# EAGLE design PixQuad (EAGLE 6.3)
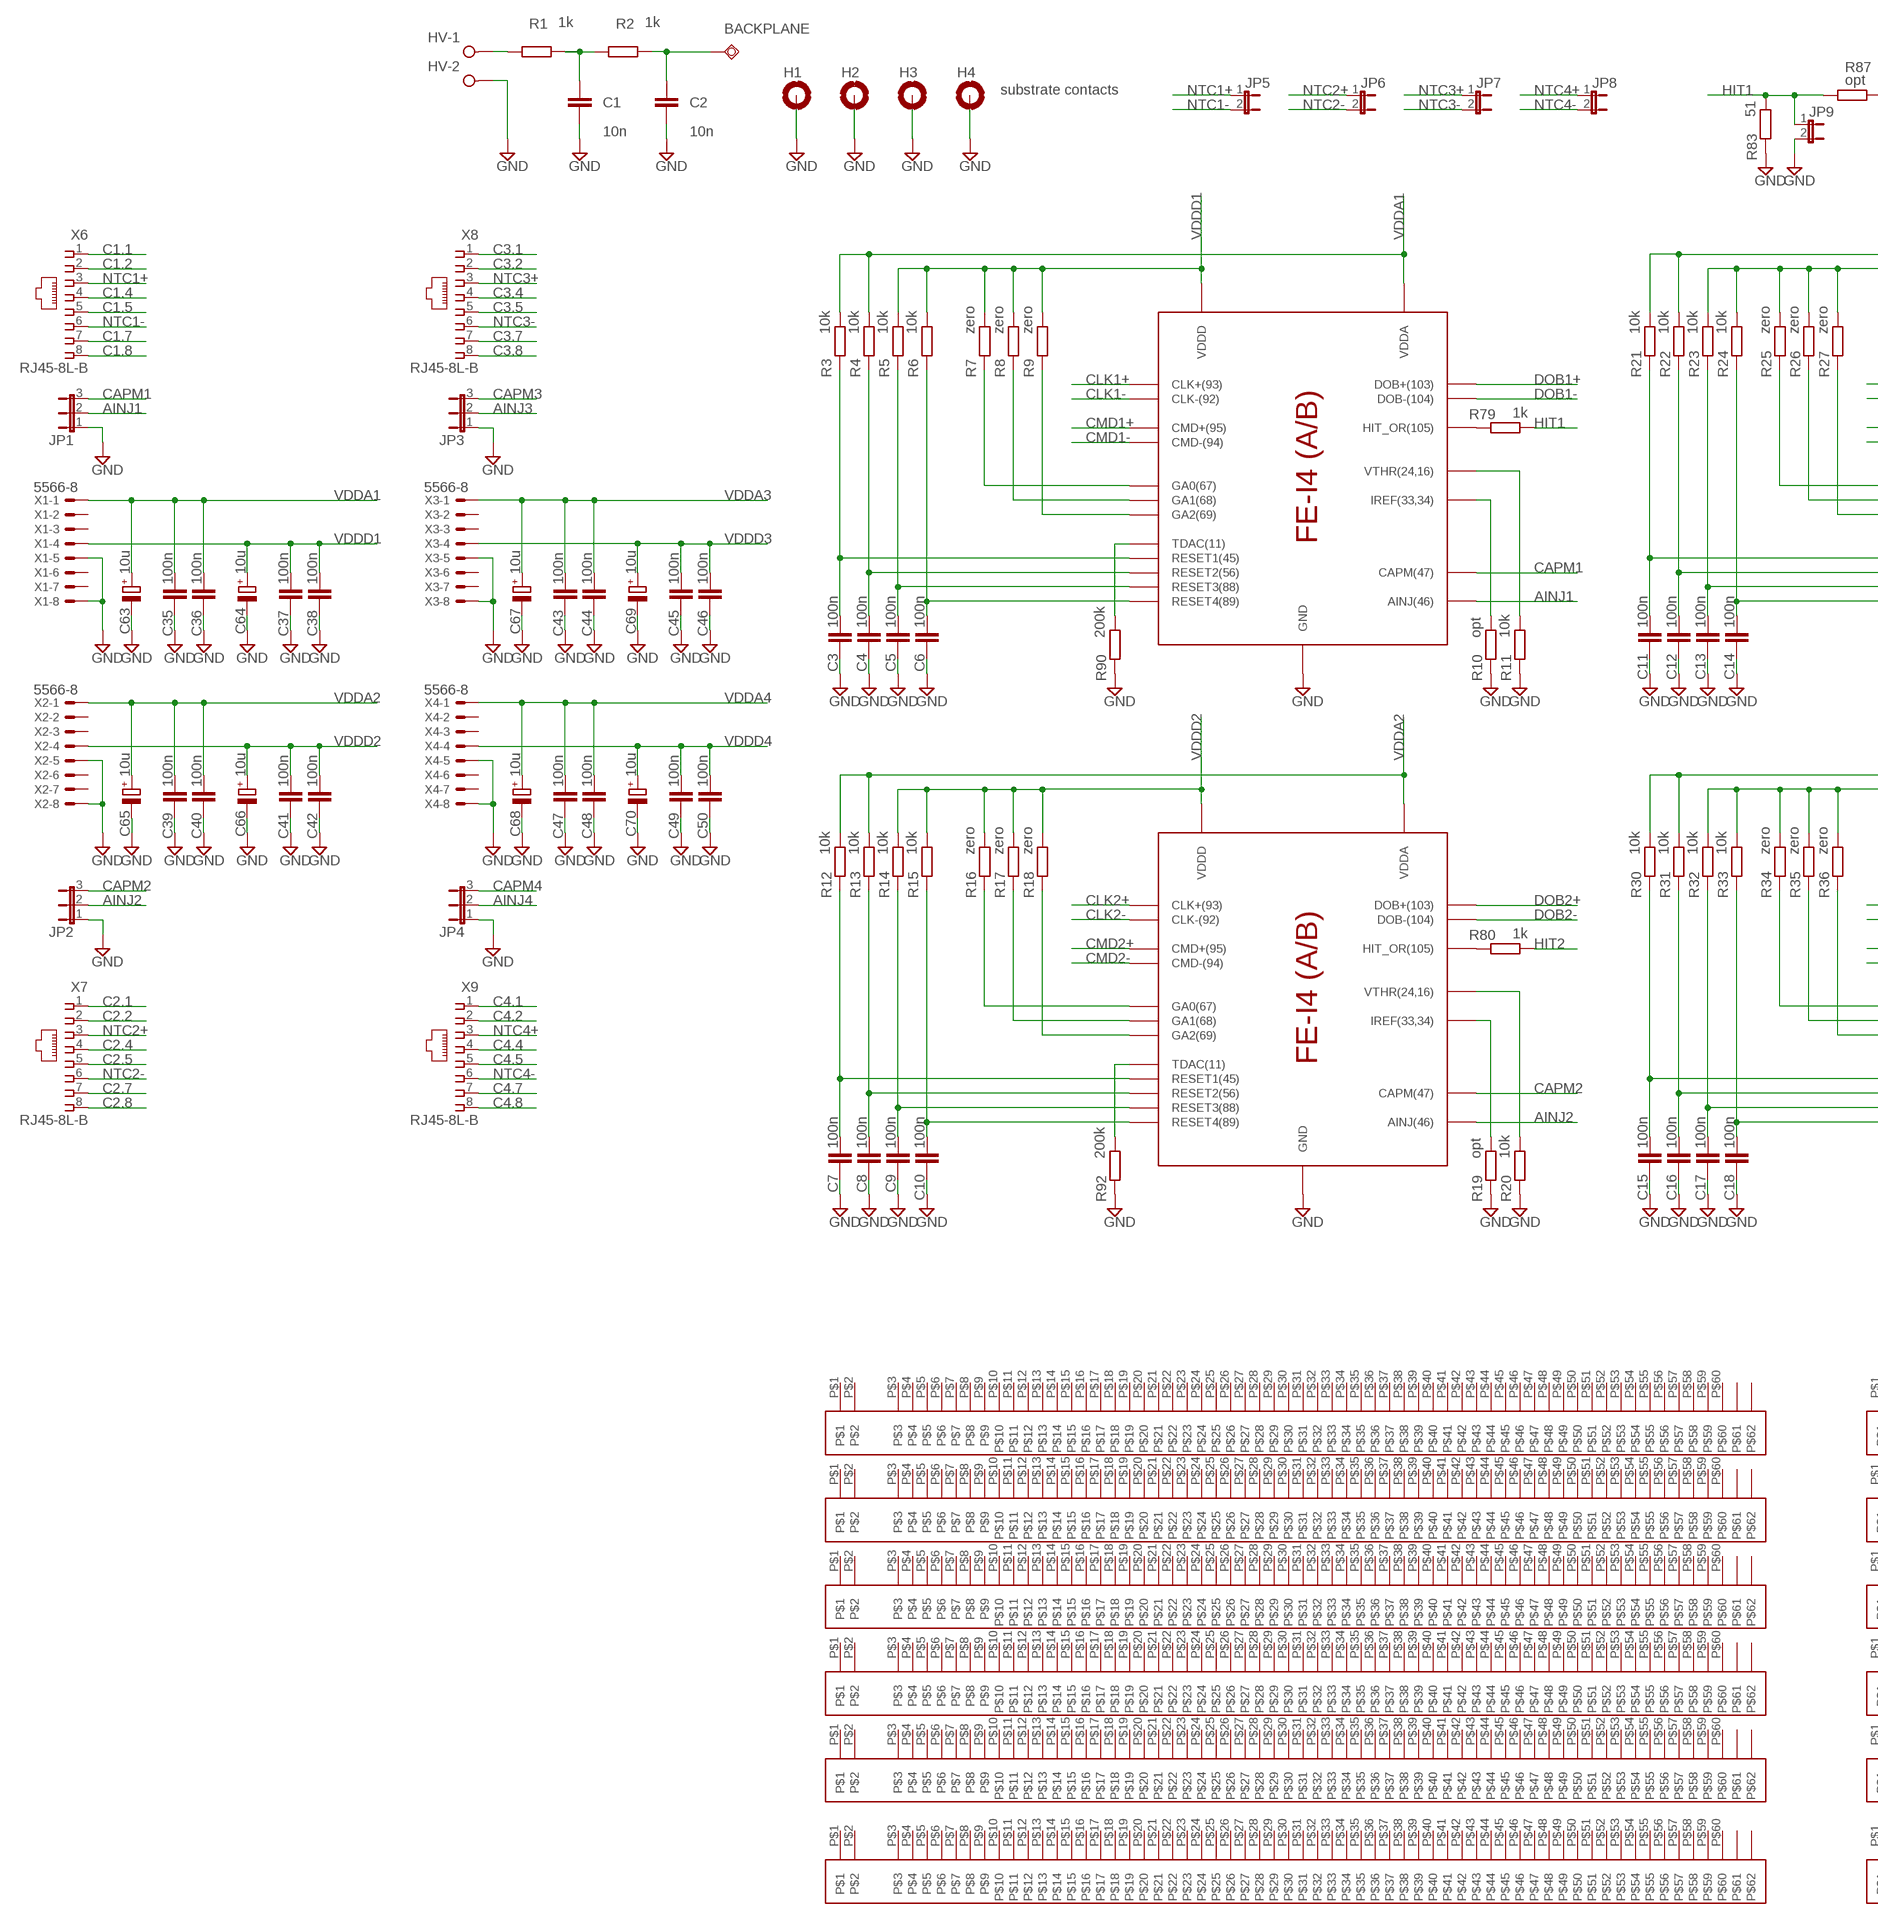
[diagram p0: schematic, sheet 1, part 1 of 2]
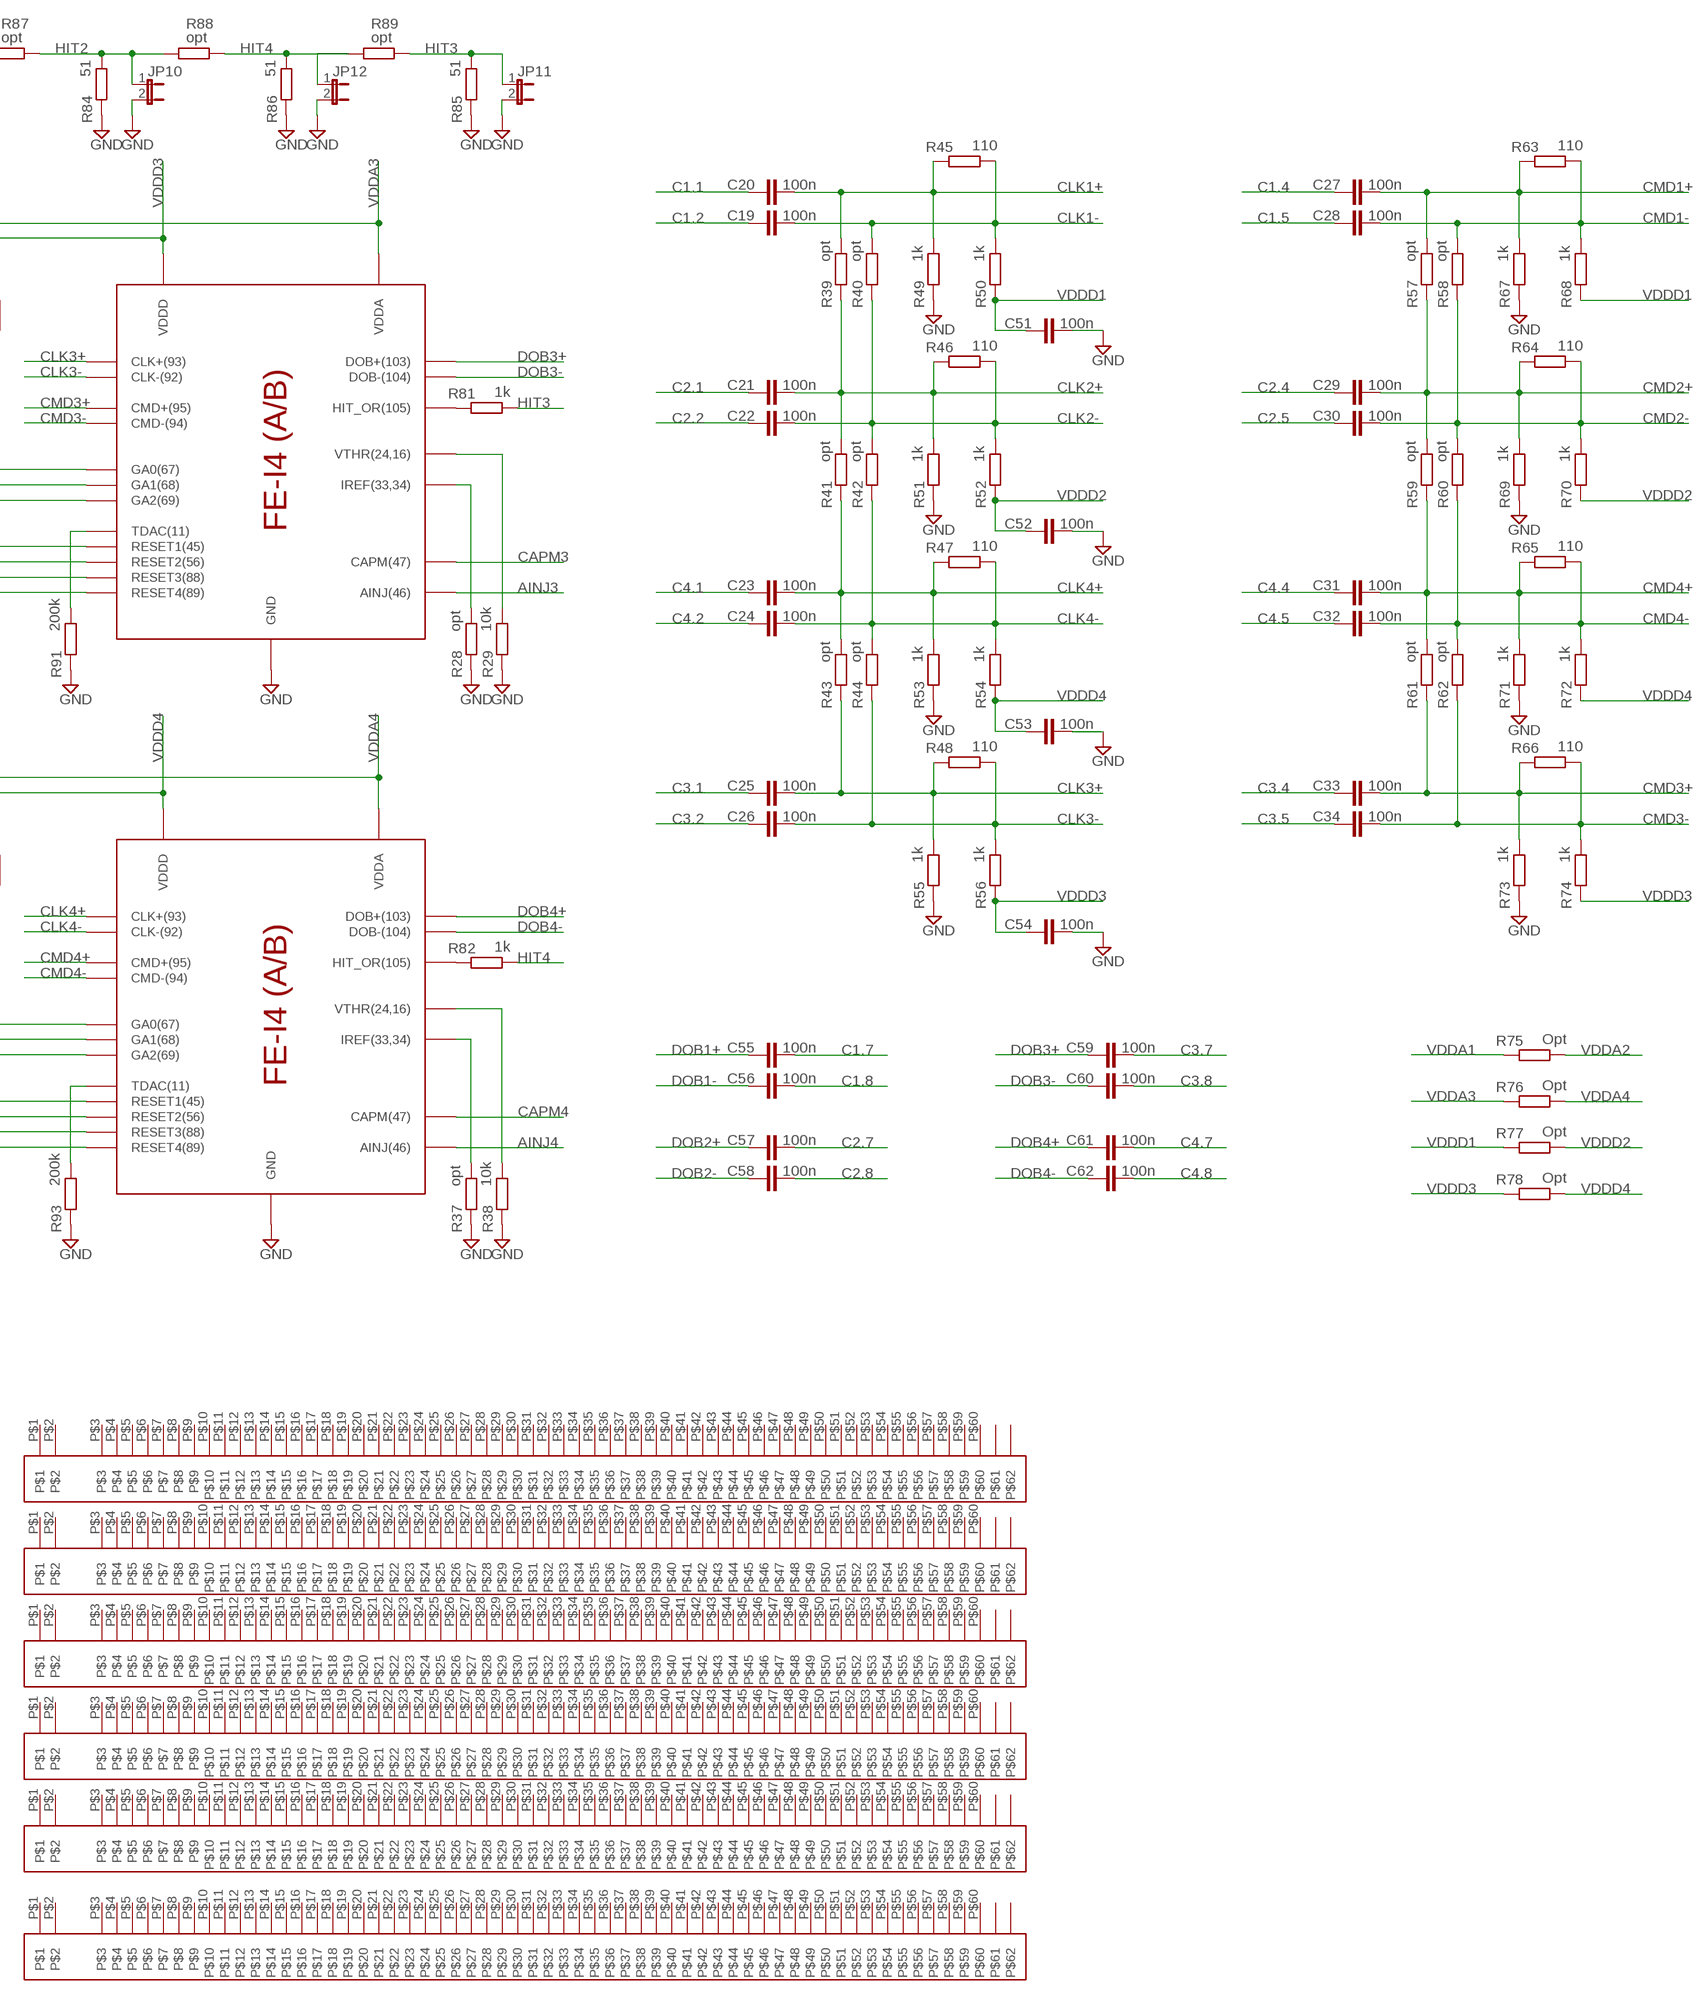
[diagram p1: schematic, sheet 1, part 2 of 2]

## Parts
BACKPLANE  TPSQTP20SQ  [TP20SQ]
C1  10n  C-EUC1210  [C1210]
C2  10n  C-EUC1210  [C1210]
C3  100n  C-EUC0402  [C0402]
C4  100n  C-EUC0402  [C0402]
C5  100n  C-EUC0402  [C0402]
C6  100n  C-EUC0402  [C0402]
C7  100n  C-EUC0402  [C0402]
C8  100n  C-EUC0402  [C0402]
C9  100n  C-EUC0402  [C0402]
C10  100n  C-EUC0402  [C0402]
C11  100n  C-EUC0402  [C0402]
C12  100n  C-EUC0402  [C0402]
C13  100n  C-EUC0402  [C0402]
C14  100n  C-EUC0402  [C0402]
C15  100n  C-EUC0402  [C0402]
C16  100n  C-EUC0402  [C0402]
C17  100n  C-EUC0402  [C0402]
C18  100n  C-EUC0402  [C0402]
C19  100n  C-EUC0402  [C0402]
C20  100n  C-EUC0402  [C0402]
C21  100n  C-EUC0402  [C0402]
C22  100n  C-EUC0402  [C0402]
C23  100n  C-EUC0402  [C0402]
C24  100n  C-EUC0402  [C0402]
C25  100n  C-EUC0402  [C0402]
C26  100n  C-EUC0402  [C0402]
C27  100n  C-EUC0402  [C0402]
C28  100n  C-EUC0402  [C0402]
C29  100n  C-EUC0402  [C0402]
C30  100n  C-EUC0402  [C0402]
C31  100n  C-EUC0402  [C0402]
C32  100n  C-EUC0402  [C0402]
C33  100n  C-EUC0402  [C0402]
C34  100n  C-EUC0402  [C0402]
C35  100n  C-EUC0402  [C0402]
C36  100n  C-EUC0402  [C0402]
C37  100n  C-EUC0402  [C0402]
C38  100n  C-EUC0402  [C0402]
C39  100n  C-EUC0402  [C0402]
C40  100n  C-EUC0402  [C0402]
C41  100n  C-EUC0402  [C0402]
C42  100n  C-EUC0402  [C0402]
C43  100n  C-EUC0402  [C0402]
C44  100n  C-EUC0402  [C0402]
C45  100n  C-EUC0402  [C0402]
C46  100n  C-EUC0402  [C0402]
C47  100n  C-EUC0402  [C0402]
C48  100n  C-EUC0402  [C0402]
C49  100n  C-EUC0402  [C0402]
C50  100n  C-EUC0402  [C0402]
C51  100n  C-EUC0402  [C0402]
C52  100n  C-EUC0402  [C0402]
C53  100n  C-EUC0402  [C0402]
C54  100n  C-EUC0402  [C0402]
C55  100n  C-EUC0402  [C0402]
C56  100n  C-EUC0402  [C0402]
C57  100n  C-EUC0402  [C0402]
C58  100n  C-EUC0402  [C0402]
C59  100n  C-EUC0402  [C0402]
C60  100n  C-EUC0402  [C0402]
C61  100n  C-EUC0402  [C0402]
C62  100n  C-EUC0402  [C0402]
C63  10u  CPOL-EUSMCA  [SMC_A]
C64  10u  CPOL-EUSMCA  [SMC_A]
C65  10u  CPOL-EUSMCA  [SMC_A]
C66  10u  CPOL-EUSMCA  [SMC_A]
C67  10u  CPOL-EUSMCA  [SMC_A]
C68  10u  CPOL-EUSMCA  [SMC_A]
C69  10u  CPOL-EUSMCA  [SMC_A]
C70  10u  CPOL-EUSMCA  [SMC_A]
H1  MOUNT-PAD-ROUND3.2  [3,2-PAD]
H2  MOUNT-PAD-ROUND3.2  [3,2-PAD]
H3  MOUNT-PAD-ROUND3.2  [3,2-PAD]
H4  substrate contacts  MOUNT-PAD-ROUND3.2  [3,2-PAD]
HV  W237-2N  [W237-2N]
JP1  JP2E  [JP2]
JP2  JP2E  [JP2]
JP3  JP2E  [JP2]
JP4  JP2E  [JP2]
JP5  JP1E  [JP1]
JP6  JP1E  [JP1]
JP7  JP1E  [JP1]
JP8  JP1E  [JP1]
JP9  JP1E  [JP1]
JP10  JP1E  [JP1]
JP11  JP1E  [JP1]
JP12  JP1E  [JP1]
R1  1k  R-EU_R1206  [R1206]
R2  1k  R-EU_R1206  [R1206]
R3  10k  R-EU_R0402  [R0402]
R4  10k  R-EU_R0402  [R0402]
R5  10k  R-EU_R0402  [R0402]
R6  10k  R-EU_R0402  [R0402]
R7  zero  R-EU_R0402  [R0402]
R8  zero  R-EU_R0402  [R0402]
R9  zero  R-EU_R0402  [R0402]
R10  opt  R-EU_R0402  [R0402]
R11  10k  R-EU_R0402  [R0402]
R12  10k  R-EU_R0402  [R0402]
R13  10k  R-EU_R0402  [R0402]
R14  10k  R-EU_R0402  [R0402]
R15  10k  R-EU_R0402  [R0402]
R16  zero  R-EU_R0402  [R0402]
R17  zero  R-EU_R0402  [R0402]
R18  zero  R-EU_R0402  [R0402]
R19  opt  R-EU_R0402  [R0402]
R20  10k  R-EU_R0402  [R0402]
R21  10k  R-EU_R0402  [R0402]
R22  10k  R-EU_R0402  [R0402]
R23  10k  R-EU_R0402  [R0402]
R24  10k  R-EU_R0402  [R0402]
R25  zero  R-EU_R0402  [R0402]
R26  zero  R-EU_R0402  [R0402]
R27  zero  R-EU_R0402  [R0402]
R28  opt  R-EU_R0402  [R0402]
R29  10k  R-EU_R0402  [R0402]
R30  10k  R-EU_R0402  [R0402]
R31  10k  R-EU_R0402  [R0402]
R32  10k  R-EU_R0402  [R0402]
R33  10k  R-EU_R0402  [R0402]
R34  zero  R-EU_R0402  [R0402]
R35  zero  R-EU_R0402  [R0402]
R36  zero  R-EU_R0402  [R0402]
R37  opt  R-EU_R0402  [R0402]
R38  10k  R-EU_R0402  [R0402]
R39  opt  R-EU_R0402  [R0402]
R40  opt  R-EU_R0402  [R0402]
R41  opt  R-EU_R0402  [R0402]
R42  opt  R-EU_R0402  [R0402]
R43  opt  R-EU_R0402  [R0402]
R44  opt  R-EU_R0402  [R0402]
R45  110  R-EU_R0402  [R0402]
R46  110  R-EU_R0402  [R0402]
R47  110  R-EU_R0402  [R0402]
R48  110  R-EU_R0402  [R0402]
R49  1k  R-EU_R0402  [R0402]
R50  1k  R-EU_R0402  [R0402]
R51  1k  R-EU_R0402  [R0402]
R52  1k  R-EU_R0402  [R0402]
R53  1k  R-EU_R0402  [R0402]
R54  1k  R-EU_R0402  [R0402]
R55  1k  R-EU_R0402  [R0402]
R56  1k  R-EU_R0402  [R0402]
R57  opt  R-EU_R0402  [R0402]
R58  opt  R-EU_R0402  [R0402]
R59  opt  R-EU_R0402  [R0402]
R60  opt  R-EU_R0402  [R0402]
R61  opt  R-EU_R0402  [R0402]
R62  opt  R-EU_R0402  [R0402]
R63  110  R-EU_R0402  [R0402]
R64  110  R-EU_R0402  [R0402]
R65  110  R-EU_R0402  [R0402]
R66  110  R-EU_R0402  [R0402]
R67  1k  R-EU_R0402  [R0402]
R68  1k  R-EU_R0402  [R0402]
R69  1k  R-EU_R0402  [R0402]
R70  1k  R-EU_R0402  [R0402]
R71  1k  R-EU_R0402  [R0402]
R72  1k  R-EU_R0402  [R0402]
R73  1k  R-EU_R0402  [R0402]
R74  1k  R-EU_R0402  [R0402]
R75  Opt  R-EU_R0402  [R0402]
R76  Opt  R-EU_R0402  [R0402]
R77  Opt  R-EU_R0402  [R0402]
R78  Opt  R-EU_R0402  [R0402]
R79  1k  R-EU_R0402  [R0402]
R80  1k  R-EU_R0402  [R0402]
R81  1k  R-EU_R0402  [R0402]
R82  1k  R-EU_R0402  [R0402]
R83  51  R-EU_R0402  [R0402]
R84  51  R-EU_R0402  [R0402]
R85  51  R-EU_R0402  [R0402]
R86  51  R-EU_R0402  [R0402]
R87  opt  R-EU_R0402  [R0402]
R88  opt  R-EU_R0402  [R0402]
R89  opt  R-EU_R0402  [R0402]
R90  200k  R-EU_R0402  [R0402]
R91  200k  R-EU_R0402  [R0402]
R92  200k  R-EU_R0402  [R0402]
R93  200k  R-EU_R0402  [R0402]
U$1  FE_I4ASIC  [FE-I4]
U$2  FE_I4ASIC  [FE-I4]
U$3  FE_I4ASIC  [FE-I4]
U$4  FE_I4ASIC  [FE-I4]
U$5  PA  [PA]
U$6  PA  [PA]
U$7  PA  [PA]
U$8  PA  [PA]
U$9  PA  [PA]
U$10  PA  [PA]
U$11  PA  [PA]
U$12  PA  [PA]
U$13  PA  [PA]
U$14  PA  [PA]
U$15  PA  [PA]
U$16  PA  [PA]
X1  5566-8  [5566-8]
X2  5566-8  [5566-8]
X3  5566-8  [5566-8]
X4  5566-8  [5566-8]
X6  RJ45-8L-B  [RJ45-NO-SHIELD]
X7  RJ45-8L-B  [RJ45-NO-SHIELD]
X8  RJ45-8L-B  [RJ45-NO-SHIELD]
X9  RJ45-8L-B  [RJ45-NO-SHIELD]

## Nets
AINJ1: JP1.2 U$1.AINJ(46)
AINJ2: JP2.2 U$2.AINJ(46)
AINJ3: JP3.2 U$3.AINJ(46)
AINJ4: JP4.2 U$4.AINJ(46)
C1.1: C20.2 X6.1
C1.2: C19.2 X6.2
C1.4: C27.2 X6.4
C1.5: C28.2 X6.5
C1.7: C55.1 X6.7
C1.8: C56.1 X6.8
C2.1: C21.2 X7.1
C2.2: C22.2 X7.2
C2.4: C29.2 X7.4
C2.5: C30.2 X7.5
C2.7: C57.1 X7.7
C2.8: C58.1 X7.8
C3.1: C25.2 X8.1
C3.2: C26.2 X8.2
C3.4: C33.2 X8.4
C3.5: C34.2 X8.5
C3.7: C59.1 X8.7
C3.8: C60.1 X8.8
C4.1: C23.2 X9.1
C4.2: C24.2 X9.2
C4.4: C31.2 X9.4
C4.5: C32.2 X9.5
C4.7: C61.1 X9.7
C4.8: C62.1 X9.8
CAPM1: JP1.3 U$1.CAPM(47)
CAPM2: JP2.3 U$2.CAPM(47)
CAPM3: JP3.3 U$3.CAPM(47)
CAPM4: JP4.3 U$4.CAPM(47)
CLK1+: C20.1 R39.2 R45.1 R49.2 U$1.CLK+(93)
CLK1-: C19.1 R40.2 R45.2 R50.2 U$1.CLK-(92)
CLK2+: C21.1 R39.1 R41.2 R46.1 R51.2 U$2.CLK+(93)
CLK2-: C22.1 R40.1 R42.2 R46.2 R52.2 U$2.CLK-(92)
CLK3+: C25.1 R43.1 R48.1 R55.2 U$3.CLK+(93)
CLK3-: C26.1 R44.1 R48.2 R56.2 U$3.CLK-(92)
CLK4+: C23.1 R41.1 R43.2 R47.1 R53.2 U$4.CLK+(93)
CLK4-: C24.1 R42.1 R44.2 R47.2 R54.2 U$4.CLK-(92)
CMD1+: C27.1 R57.2 R63.1 R67.2 U$1.CMD+(95)
CMD1-: C28.1 R58.2 R63.2 R68.2 U$1.CMD-(94)
CMD2+: C29.1 R57.1 R59.2 R64.1 R69.2 U$2.CMD+(95)
CMD2-: C30.1 R58.1 R60.2 R64.2 R70.2 U$2.CMD-(94)
CMD3+: C33.1 R61.1 R66.1 R73.2 U$3.CMD+(95)
CMD3-: C34.1 R62.1 R66.2 R74.2 U$3.CMD-(94)
CMD4+: C31.1 R59.1 R61.2 R65.1 R71.2 U$4.CMD+(95)
CMD4-: C32.1 R60.1 R62.2 R65.2 R72.2 U$4.CMD-(94)
DOB1+: C55.2 U$1.DOB+(103)
DOB1-: C56.2 U$1.DOB-(104)
DOB2+: C57.2 U$2.DOB+(103)
DOB2-: C58.2 U$2.DOB-(104)
DOB3+: C59.2 U$3.DOB+(103)
DOB3-: C60.2 U$3.DOB-(104)
DOB4+: C61.2 U$4.DOB+(103)
DOB4-: C62.2 U$4.DOB-(104)
GND: C1.2 C2.2 C3.2 C4.2 C5.2 C6.2 C7.2 C8.2 C9.2 C10.2 C11.2 C12.2 C13.2 C14.2 C15.2 C16.2 C17.2 C18.2 C35.2 C36.2 C37.2 C38.2 C39.2 C40.2 C41.2 C42.2 C43.2 C44.2 C45.2 C46.2 C47.2 C48.2 C49.2 C50.2 C51.1 C52.1 C53.1 C54.1 C63.- C64.- C65.- C66.- C67.- C68.- C69.- C70.- H1.B3,2(MOUNT) H2.B3,2(MOUNT) H3.B3,2(MOUNT) H4.B3,2(MOUNT) HV.2 JP1.1 JP2.1 JP3.1 JP4.1 JP9.2 JP10.2 JP11.2 JP12.2 R10.1 R11.1 R19.1 R20.1 R28.1 R29.1 R37.1 R38.1 R49.1 R51.1 R53.1 R55.1 R67.1 R69.1 R71.1 R73.1 R83.1 R84.1 R85.1 R86.1 R90.1 R91.1 R92.1 R93.1 U$1.GND U$2.GND U$3.GND U$4.GND X1.5 X1.8 X2.5 X2.8 X3.5 X3.8 X4.5 X4.8
HIT1: JP9.1 R79.2 R83.2 R87.2
HIT2: JP10.1 R80.2 R84.2 R87.1 R88.2
HIT3: JP11.1 R81.2 R85.2 R89.1
HIT4: JP12.1 R82.2 R86.2 R88.1 R89.2
N$1: BACKPLANE.TP C2.1 R2.2
N$2: C1.1 R1.2 R2.1
N$3: HV.1 R1.1
N$4: C3.1 R3.1 U$1.RESET1(45)
N$5: C4.1 R4.1 U$1.RESET2(56)
N$6: C5.1 R5.1 U$1.RESET3(88)
N$7: C6.1 R6.1 U$1.RESET4(89)
N$8: R7.1 U$1.GA0(67)
N$9: R8.1 U$1.GA1(68)
N$10: R9.1 U$1.GA2(69)
N$11: R10.2 U$1.IREF(33,34)
N$12: R11.2 U$1.VTHR(24,16)
N$13: R79.1 U$1.P$1(HIT_OR(105))
N$14: R16.1 U$2.GA0(67)
N$15: R17.1 U$2.GA1(68)
N$16: R18.1 U$2.GA2(69)
N$17: C7.1 R12.1 U$2.RESET1(45)
N$18: C8.1 R13.1 U$2.RESET2(56)
N$19: C9.1 R14.1 U$2.RESET3(88)
N$20: C10.1 R15.1 U$2.RESET4(89)
N$21: R80.1 U$2.P$1(HIT_OR(105))
N$22: R81.1 U$3.P$1(HIT_OR(105))
N$23: R82.1 U$4.P$1(HIT_OR(105))
N$24: R90.2 U$1.TDAC(11)
N$25: R19.2 U$2.IREF(33,34)
N$26: R20.2 U$2.VTHR(24,16)
N$27: R91.2 U$3.TDAC(11)
N$28: R92.2 U$2.TDAC(11)
N$29: R93.2 U$4.TDAC(11)
N$50: R27.1 U$3.GA2(69)
N$56: R28.2 U$3.IREF(33,34)
N$57: R26.1 U$3.GA1(68)
N$58: R25.1 U$3.GA0(67)
N$59: C11.1 R21.1 U$3.RESET1(45)
N$60: C12.1 R22.1 U$3.RESET2(56)
N$61: C13.1 R23.1 U$3.RESET3(88)
N$62: C14.1 R24.1 U$3.RESET4(89)
N$64: R29.2 U$3.VTHR(24,16)
N$73: R34.1 U$4.GA0(67)
N$74: R35.1 U$4.GA1(68)
N$75: R36.1 U$4.GA2(69)
N$76: C15.1 R30.1 U$4.RESET1(45)
N$77: C16.1 R31.1 U$4.RESET2(56)
N$78: C17.1 R32.1 U$4.RESET3(88)
N$79: C18.1 R33.1 U$4.RESET4(89)
N$80: R37.2 U$4.IREF(33,34)
N$81: R38.2 U$4.VTHR(24,16)
NTC1+: JP5.1 X6.3
NTC1-: JP5.2 X6.6
NTC2+: JP6.1 X7.3
NTC2-: JP6.2 X7.6
NTC3+: JP7.1 X8.3
NTC3-: JP7.2 X8.6
NTC4+: JP8.1 X9.3
NTC4-: JP8.2 X9.6
VDDA1: C35.1 C36.1 C63.+ R3.2 R4.2 R75.1 U$1.VDDA X1.1
VDDA2: C39.1 C40.1 C65.+ R12.2 R13.2 R75.2 U$2.VDDA X2.1
VDDA3: C43.1 C44.1 C67.+ R21.2 R22.2 R76.1 U$3.VDDA X3.1
VDDA4: C47.1 C48.1 C68.+ R30.2 R31.2 R76.2 U$4.VDDA X4.1
VDDD1: C37.1 C38.1 C51.2 C64.+ R5.2 R6.2 R7.2 R8.2 R9.2 R50.1 R68.1 R77.1 U$1.VDDD X1.4
VDDD2: C41.1 C42.1 C52.2 C66.+ R14.2 R15.2 R16.2 R17.2 R18.2 R52.1 R70.1 R77.2 U$2.VDDD X2.4
VDDD3: C45.1 C46.1 C54.2 C69.+ R23.2 R24.2 R25.2 R26.2 R27.2 R56.1 R74.1 R78.1 U$3.VDDD X3.4
VDDD4: C49.1 C50.1 C53.2 C70.+ R32.2 R33.2 R34.2 R35.2 R36.2 R54.1 R72.1 R78.2 U$4.VDDD X4.4
Unconnected: U$5.P$1 U$5.P$2 U$5.P$3 U$5.P$4 U$5.P$5 U$5.P$6 U$5.P$7 U$5.P$8 U$5.P$9 U$5.P$10 U$5.P$11 U$5.P$12 U$5.P$13 U$5.P$14 U$5.P$15 U$5.P$16 U$5.P$17 U$5.P$18 U$5.P$19 U$5.P$20 U$5.P$21 U$5.P$22 U$5.P$23 U$5.P$24 U$5.P$25 U$5.P$26 U$5.P$27 U$5.P$28 U$5.P$29 U$5.P$30 U$5.P$31 U$5.P$32 U$5.P$33 U$5.P$34 U$5.P$35 U$5.P$36 U$5.P$37 U$5.P$38 U$5.P$39 U$5.P$40 U$5.P$41 U$5.P$42 U$5.P$43 U$5.P$44 U$5.P$45 U$5.P$46 U$5.P$47 U$5.P$48 U$5.P$49 U$5.P$50 U$5.P$51 U$5.P$52 U$5.P$53 U$5.P$54 U$5.P$55 U$5.P$56 U$5.P$57 U$5.P$58 U$5.P$59 U$5.P$60 U$5.P$61 U$5.P$62 U$6.P$1 U$6.P$2 U$6.P$3 U$6.P$4 U$6.P$5 U$6.P$6 U$6.P$7 U$6.P$8 U$6.P$9 U$6.P$10 U$6.P$11 U$6.P$12 U$6.P$13 U$6.P$14 U$6.P$15 U$6.P$16 U$6.P$17 U$6.P$18 U$6.P$19 U$6.P$20 U$6.P$21 U$6.P$22 U$6.P$23 U$6.P$24 U$6.P$25 U$6.P$26 U$6.P$27 U$6.P$28 U$6.P$29 U$6.P$30 U$6.P$31 U$6.P$32 U$6.P$33 U$6.P$34 U$6.P$35 U$6.P$36 U$6.P$37 U$6.P$38 U$6.P$39 U$6.P$40 U$6.P$41 U$6.P$42 U$6.P$43 U$6.P$44 U$6.P$45 U$6.P$46 U$6.P$47 U$6.P$48 U$6.P$49 U$6.P$50 U$6.P$51 U$6.P$52 U$6.P$53 U$6.P$54 U$6.P$55 U$6.P$56 U$6.P$57 U$6.P$58 U$6.P$59 U$6.P$60 U$6.P$61 U$6.P$62 U$7.P$1 U$7.P$2 U$7.P$3 U$7.P$4 U$7.P$5 U$7.P$6 U$7.P$7 U$7.P$8 U$7.P$9 U$7.P$10 U$7.P$11 U$7.P$12 U$7.P$13 U$7.P$14 U$7.P$15 U$7.P$16 U$7.P$17 U$7.P$18 U$7.P$19 U$7.P$20 U$7.P$21 U$7.P$22 U$7.P$23 U$7.P$24 U$7.P$25 U$7.P$26 U$7.P$27 U$7.P$28 U$7.P$29 U$7.P$30 U$7.P$31 U$7.P$32 U$7.P$33 U$7.P$34 U$7.P$35 U$7.P$36 U$7.P$37 U$7.P$38 U$7.P$39 U$7.P$40 U$7.P$41 U$7.P$42 U$7.P$43 U$7.P$44 U$7.P$45 U$7.P$46 U$7.P$47 U$7.P$48 U$7.P$49 U$7.P$50 U$7.P$51 U$7.P$52 U$7.P$53 U$7.P$54 U$7.P$55 U$7.P$56 U$7.P$57 U$7.P$58 U$7.P$59 U$7.P$60 U$7.P$61 U$7.P$62 U$8.P$1 U$8.P$2 U$8.P$3 U$8.P$4 U$8.P$5 U$8.P$6 U$8.P$7 U$8.P$8 U$8.P$9 U$8.P$10 U$8.P$11 U$8.P$12 U$8.P$13 U$8.P$14 U$8.P$15 U$8.P$16 U$8.P$17 U$8.P$18 U$8.P$19 U$8.P$20 U$8.P$21 U$8.P$22 U$8.P$23 U$8.P$24 U$8.P$25 U$8.P$26 U$8.P$27 U$8.P$28 U$8.P$29 U$8.P$30 U$8.P$31 U$8.P$32 U$8.P$33 U$8.P$34 U$8.P$35 U$8.P$36 U$8.P$37 U$8.P$38 U$8.P$39 U$8.P$40 U$8.P$41 U$8.P$42 U$8.P$43 U$8.P$44 U$8.P$45 U$8.P$46 U$8.P$47 U$8.P$48 U$8.P$49 U$8.P$50 U$8.P$51 U$8.P$52 U$8.P$53 U$8.P$54 U$8.P$55 U$8.P$56 U$8.P$57 U$8.P$58 U$8.P$59 U$8.P$60 U$8.P$61 U$8.P$62 U$9.P$1 U$9.P$2 U$9.P$3 U$9.P$4 U$9.P$5 U$9.P$6 U$9.P$7 U$9.P$8 U$9.P$9 U$9.P$10 U$9.P$11 U$9.P$12 U$9.P$13 U$9.P$14 U$9.P$15 U$9.P$16 U$9.P$17 U$9.P$18 U$9.P$19 U$9.P$20 U$9.P$21 U$9.P$22 U$9.P$23 U$9.P$24 U$9.P$25 U$9.P$26 U$9.P$27 U$9.P$28 U$9.P$29 U$9.P$30 U$9.P$31 U$9.P$32 U$9.P$33 U$9.P$34 U$9.P$35 U$9.P$36 U$9.P$37 U$9.P$38 U$9.P$39 U$9.P$40 U$9.P$41 U$9.P$42 U$9.P$43 U$9.P$44 U$9.P$45 U$9.P$46 U$9.P$47 U$9.P$48 U$9.P$49 U$9.P$50 U$9.P$51 U$9.P$52 U$9.P$53 U$9.P$54 U$9.P$55 U$9.P$56 U$9.P$57 U$9.P$58 U$9.P$59 U$9.P$60 U$9.P$61 U$9.P$62 U$10.P$1 U$10.P$2 U$10.P$3 U$10.P$4 U$10.P$5 U$10.P$6 U$10.P$7 U$10.P$8 U$10.P$9 U$10.P$10 U$10.P$11 U$10.P$12 U$10.P$13 U$10.P$14 U$10.P$15 U$10.P$16 U$10.P$17 U$10.P$18 U$10.P$19 U$10.P$20 U$10.P$21 U$10.P$22 U$10.P$23 U$10.P$24 U$10.P$25 U$10.P$26 U$10.P$27 U$10.P$28 U$10.P$29 U$10.P$30 U$10.P$31 U$10.P$32 U$10.P$33 U$10.P$34 U$10.P$35 U$10.P$36 U$10.P$37 U$10.P$38 U$10.P$39 U$10.P$40 U$10.P$41 U$10.P$42 U$10.P$43 U$10.P$44 U$10.P$45 U$10.P$46 U$10.P$47 U$10.P$48 U$10.P$49 U$10.P$50 U$10.P$51 U$10.P$52 U$10.P$53 U$10.P$54 U$10.P$55 U$10.P$56 U$10.P$57 U$10.P$58 U$10.P$59 U$10.P$60 U$10.P$61 U$10.P$62 U$11.P$1 U$11.P$2 U$11.P$3 U$11.P$4 U$11.P$5 U$11.P$6 U$11.P$7 U$11.P$8 U$11.P$9 U$11.P$10 U$11.P$11 U$11.P$12 U$11.P$13 U$11.P$14 U$11.P$15 U$11.P$16 U$11.P$17 U$11.P$18 U$11.P$19 U$11.P$20 U$11.P$21 U$11.P$22 U$11.P$23 U$11.P$24 U$11.P$25 U$11.P$26 U$11.P$27 U$11.P$28 U$11.P$29 U$11.P$30 U$11.P$31 U$11.P$32 U$11.P$33 U$11.P$34 U$11.P$35 U$11.P$36 U$11.P$37 U$11.P$38 U$11.P$39 U$11.P$40 U$11.P$41 U$11.P$42 U$11.P$43 U$11.P$44 U$11.P$45 U$11.P$46 U$11.P$47 U$11.P$48 U$11.P$49 U$11.P$50 U$11.P$51 U$11.P$52 U$11.P$53 U$11.P$54 U$11.P$55 U$11.P$56 U$11.P$57 U$11.P$58 U$11.P$59 U$11.P$60 U$11.P$61 U$11.P$62 U$12.P$1 U$12.P$2 U$12.P$3 U$12.P$4 U$12.P$5 U$12.P$6 U$12.P$7 U$12.P$8 U$12.P$9 U$12.P$10 U$12.P$11 U$12.P$12 U$12.P$13 U$12.P$14 U$12.P$15 U$12.P$16 U$12.P$17 U$12.P$18 U$12.P$19 U$12.P$20 U$12.P$21 U$12.P$22 U$12.P$23 U$12.P$24 U$12.P$25 U$12.P$26 U$12.P$27 U$12.P$28 U$12.P$29 U$12.P$30 U$12.P$31 U$12.P$32 U$12.P$33 U$12.P$34 U$12.P$35 U$12.P$36 U$12.P$37 U$12.P$38 U$12.P$39 U$12.P$40 U$12.P$41 U$12.P$42 U$12.P$43 U$12.P$44 U$12.P$45 U$12.P$46 U$12.P$47 U$12.P$48 U$12.P$49 U$12.P$50 U$12.P$51 U$12.P$52 U$12.P$53 U$12.P$54 U$12.P$55 U$12.P$56 U$12.P$57 U$12.P$58 U$12.P$59 U$12.P$60 U$12.P$61 U$12.P$62 U$13.P$1 U$13.P$2 U$13.P$3 U$13.P$4 U$13.P$5 U$13.P$6 U$13.P$7 U$13.P$8 U$13.P$9 U$13.P$10 U$13.P$11 U$13.P$12 U$13.P$13 U$13.P$14 U$13.P$15 U$13.P$16 U$13.P$17 U$13.P$18 U$13.P$19 U$13.P$20 U$13.P$21 U$13.P$22 U$13.P$23 U$13.P$24 U$13.P$25 U$13.P$26 U$13.P$27 U$13.P$28 U$13.P$29 U$13.P$30 U$13.P$31 U$13.P$32 U$13.P$33 U$13.P$34 U$13.P$35 U$13.P$36 U$13.P$37 U$13.P$38 U$13.P$39 U$13.P$40 U$13.P$41 U$13.P$42 U$13.P$43 U$13.P$44 U$13.P$45 U$13.P$46 U$13.P$47 U$13.P$48 U$13.P$49 U$13.P$50 U$13.P$51 U$13.P$52 U$13.P$53 U$13.P$54 U$13.P$55 U$13.P$56 U$13.P$57 U$13.P$58 U$13.P$59 U$13.P$60 U$13.P$61 U$13.P$62 U$14.P$1 U$14.P$2 U$14.P$3 U$14.P$4 U$14.P$5 U$14.P$6 U$14.P$7 U$14.P$8 U$14.P$9 U$14.P$10 U$14.P$11 U$14.P$12 U$14.P$13 U$14.P$14 U$14.P$15 U$14.P$16 U$14.P$17 U$14.P$18 U$14.P$19 U$14.P$20 U$14.P$21 U$14.P$22 U$14.P$23 U$14.P$24 U$14.P$25 U$14.P$26 U$14.P$27 U$14.P$28 U$14.P$29 U$14.P$30 U$14.P$31 U$14.P$32 U$14.P$33 U$14.P$34 U$14.P$35 U$14.P$36 U$14.P$37 U$14.P$38 U$14.P$39 U$14.P$40 U$14.P$41 U$14.P$42 U$14.P$43 U$14.P$44 U$14.P$45 U$14.P$46 U$14.P$47 U$14.P$48 U$14.P$49 U$14.P$50 U$14.P$51 U$14.P$52 U$14.P$53 U$14.P$54 U$14.P$55 U$14.P$56 U$14.P$57 U$14.P$58 U$14.P$59 U$14.P$60 U$14.P$61 U$14.P$62 U$15.P$1 U$15.P$2 U$15.P$3 U$15.P$4 U$15.P$5 U$15.P$6 U$15.P$7 U$15.P$8 U$15.P$9 U$15.P$10 U$15.P$11 U$15.P$12 U$15.P$13 U$15.P$14 U$15.P$15 U$15.P$16 U$15.P$17 U$15.P$18 U$15.P$19 U$15.P$20 U$15.P$21 U$15.P$22 U$15.P$23 U$15.P$24 U$15.P$25 U$15.P$26 U$15.P$27 U$15.P$28 U$15.P$29 U$15.P$30 U$15.P$31 U$15.P$32 U$15.P$33 U$15.P$34 U$15.P$35 U$15.P$36 U$15.P$37 U$15.P$38 U$15.P$39 U$15.P$40 U$15.P$41 U$15.P$42 U$15.P$43 U$15.P$44 U$15.P$45 U$15.P$46 U$15.P$47 U$15.P$48 U$15.P$49 U$15.P$50 U$15.P$51 U$15.P$52 U$15.P$53 U$15.P$54 U$15.P$55 U$15.P$56 U$15.P$57 U$15.P$58 U$15.P$59 U$15.P$60 U$15.P$61 U$15.P$62 U$16.P$1 U$16.P$2 U$16.P$3 U$16.P$4 U$16.P$5 U$16.P$6 U$16.P$7 U$16.P$8 U$16.P$9 U$16.P$10 U$16.P$11 U$16.P$12 U$16.P$13 U$16.P$14 U$16.P$15 U$16.P$16 U$16.P$17 U$16.P$18 U$16.P$19 U$16.P$20 U$16.P$21 U$16.P$22 U$16.P$23 U$16.P$24 U$16.P$25 U$16.P$26 U$16.P$27 U$16.P$28 U$16.P$29 U$16.P$30 U$16.P$31 U$16.P$32 U$16.P$33 U$16.P$34 U$16.P$35 U$16.P$36 U$16.P$37 U$16.P$38 U$16.P$39 U$16.P$40 U$16.P$41 U$16.P$42 U$16.P$43 U$16.P$44 U$16.P$45 U$16.P$46 U$16.P$47 U$16.P$48 U$16.P$49 U$16.P$50 U$16.P$51 U$16.P$52 U$16.P$53 U$16.P$54 U$16.P$55 U$16.P$56 U$16.P$57 U$16.P$58 U$16.P$59 U$16.P$60 U$16.P$61 U$16.P$62 X1.2 X1.3 X1.6 X1.7 X2.2 X2.3 X2.6 X2.7 X3.2 X3.3 X3.6 X3.7 X4.2 X4.3 X4.6 X4.7

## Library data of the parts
BACKPLANE = testpad:TPSQ: Test pad
C1-C62 = rcl:C-EU: CAPACITOR, European symbol
C63-C70 = rcl:CPOL-EU: POLARIZED CAPACITOR, European symbol
H1-H4 = holes:MOUNT-PAD-ROUND: MOUNTING PAD, round
HV = con-wago-508:W237-2N: WAGO SREW CLAMP; OC_FARNELL: unknown; OC_NEWARK: unknown
JP1-JP4 = jumper:JP2E: JUMPER
JP5-JP12 = jumper:JP1E: JUMPER
R1-R93 = rcl:R-EU_: RESISTOR, European symbol
U$1-U$4 = FE-I4:FE_I4
U$5-U$16 = FE-I4:PA
X1-X4 = FE-I4:5566-8: Mini FIT connector 8 pol Source: http://www.molex.com; OC_FARNELL: unknown; OC_NEWARK: unknown
X6-X9 = con-tycoelectronics:RJ45: CORCOM Modular RJ Jacks No Shield Source: www.tycoelectronics.com .. ENG_DS_1654001_1099_RJ_L_0507.pdf; MF: TYCO ELECTRONICS; MPN: RJ45-8L-B; OC_FARNELL: 1279843; OC_NEWARK: 52K4445

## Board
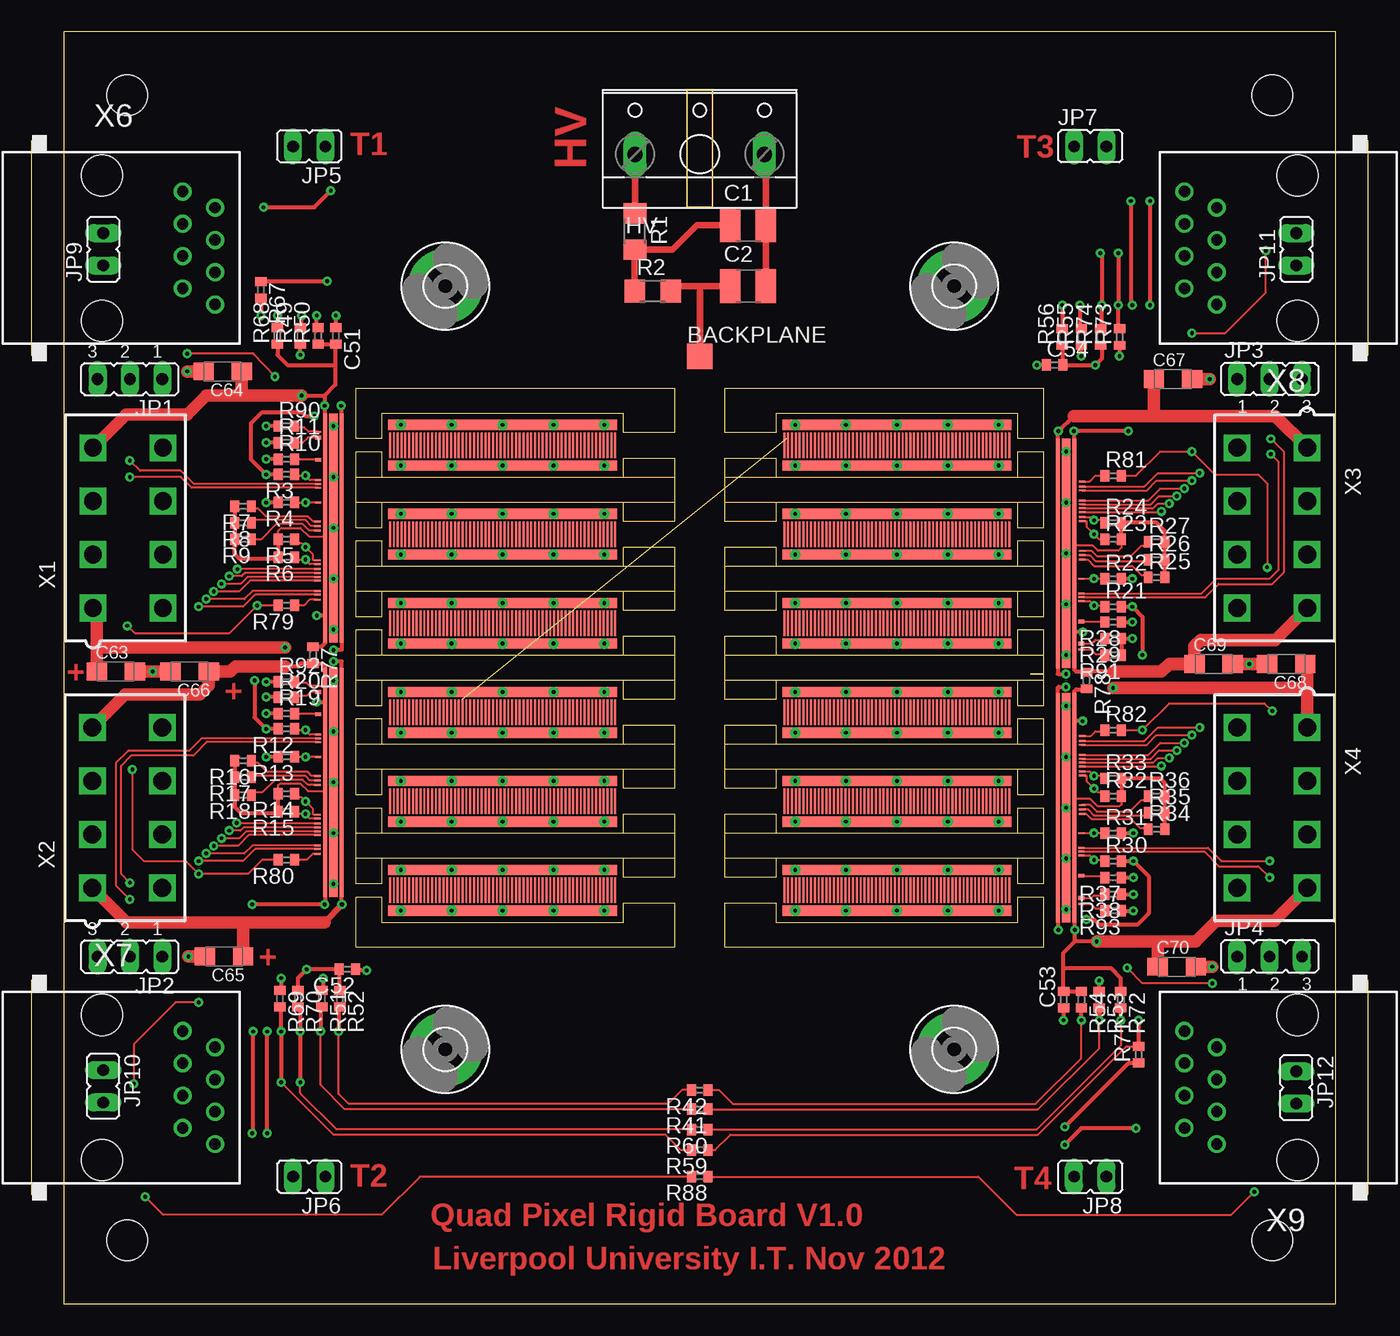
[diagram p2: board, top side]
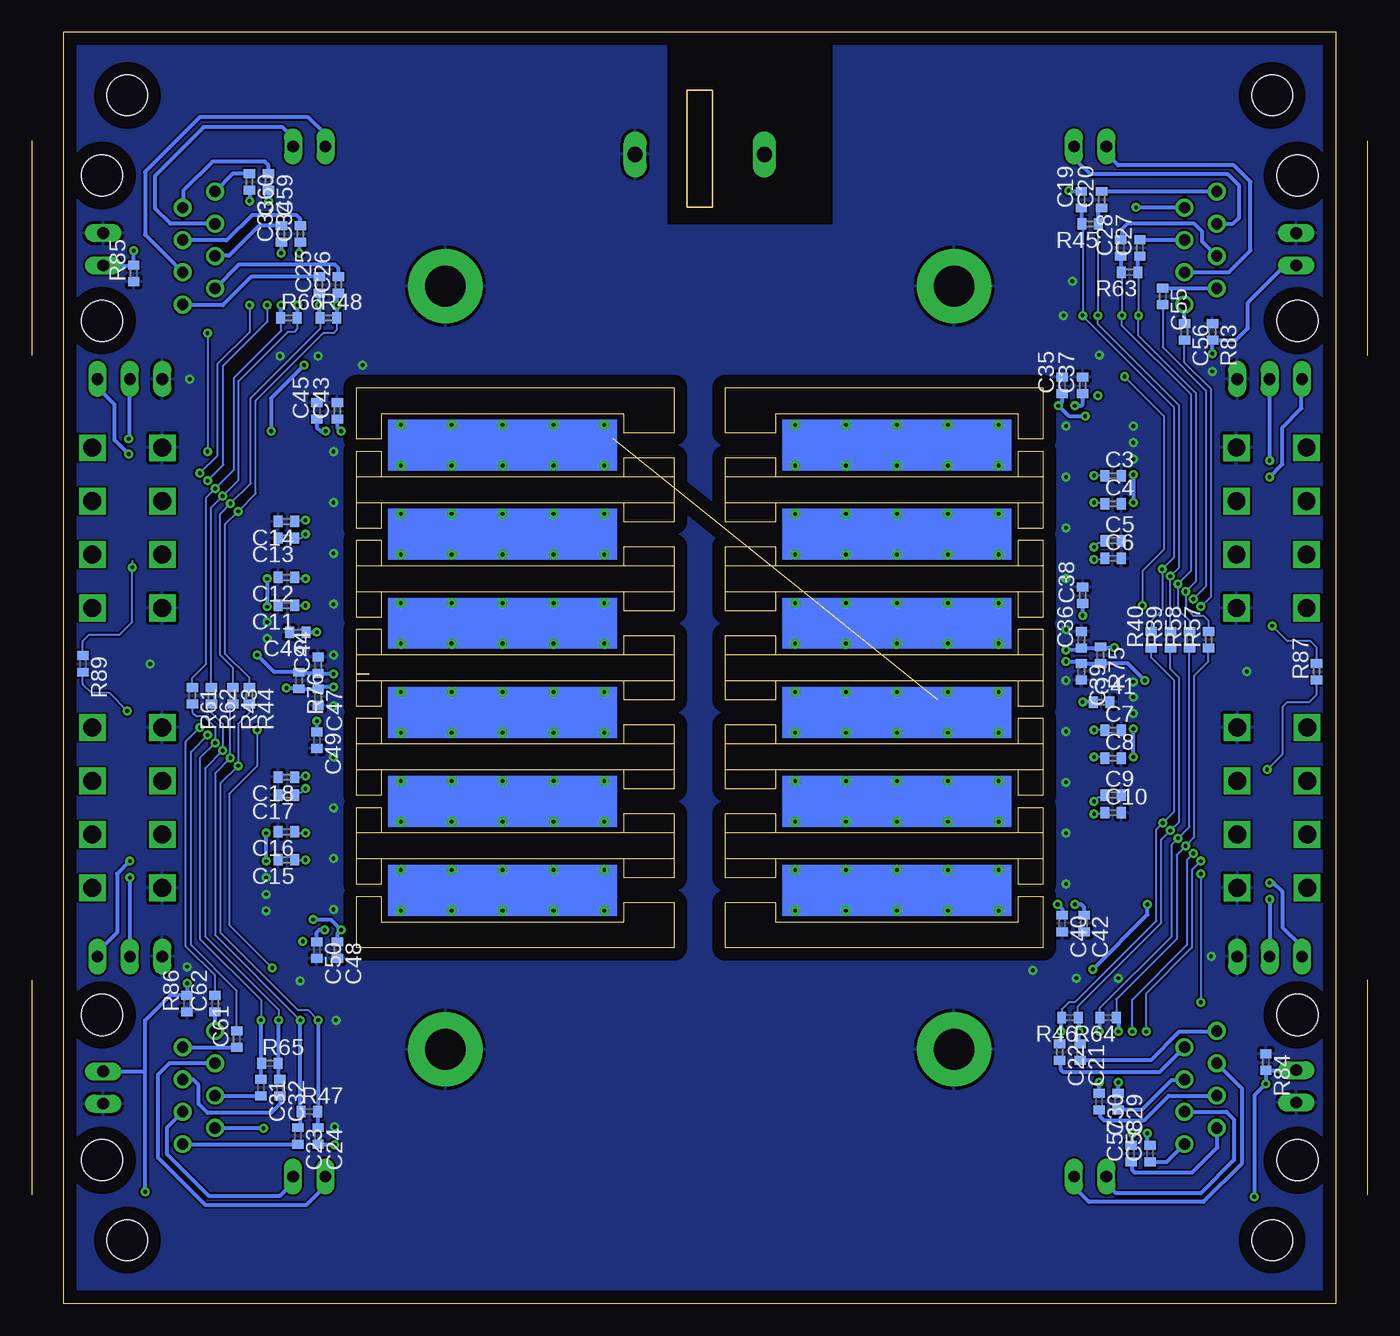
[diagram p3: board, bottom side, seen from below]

Size 105.02 x 100 mm. Coordinates in mm from the lower left corner, seen from the top.
Outline: 2.51,0 102.51,0 102.51,100 2.51,100 2.51,0
Copper layers (1+2*15+16): Top 0.035mm / dielectric 1.5mm / Route2 0.035mm / dielectric 0.15mm / Route15 0.035mm / dielectric 0.2mm / Bottom 0.035mm
Design rules "default *": minimum track width 10mil, minimum drill 24mil, track to track 6mil, track to pad 6mil, pad to pad 6mil, via to via 6mil, smd to smd 6mil, copper to edge 40mil, drill to drill 8mil, minimum pad ring 10mil, minimum via ring 8mil, stop-mask expansion 4mil, vias tented up to drill 0mil, thermal gap 10mil
Holes 3.2 mm at 7.51,5 7.51,95 97.51,95 97.51,5

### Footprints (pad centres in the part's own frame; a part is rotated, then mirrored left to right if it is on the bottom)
TP20SQ = smd 2 x 2: TP 0,0
C1210 = smd 1.6 x 2.7: 1 -1.4,0; 2 1.4,0
C0402 = smd 0.7 x 0.9: 1 -0.65,0; 2 0.65,0
SMC_A = smd 1.6 x 1.4: + -1.5,0; - 1.5,0
3,2-PAD = drill 3.2 pad 5.842: B3,2 0,0
W237-2N = drill 1.194 long: 1 -5.08,-0.635; 2 5.08,-0.635
JP2 = drill 0.914 long: 1 -2.54,0; 2 0,0; 3 2.54,0
JP1 = drill 0.914 long: 1 0,-1.27; 2 0,1.27
R1206 = smd 1.6 x 1.803: 1 -1.422,0; 2 1.422,0
R0402 = smd 0.7 x 0.9: 1 -0.65,0; 2 0.65,0
FE-I4 = smd 0.15 x 0.5: AINJ(46) -4.45,-2; CAPM(47) -4.15,-2; CLK+(93) 2.55,-2.05; CLK-(92) 2.25,-2.05; CMD+(95) 3.15,-2.05; CMD-(94) 2.85,-2.05; DOB+(103) 3.95,-2.05; DOB-(104) 4.25,-2.05; GA0(67) -1.5,-2.05; GA1(68) -1.15,-2.05; GA2(69) -0.8,-2.05; P$1 4.65,-2.05; RESET1(45) -4.75,-2; RESET2(56) -3,-2; RESET3(88) 1.55,-2.05; RESET4(89) 1.85,-2.05; TDAC(11) -8.55,-2 | smd 18 x 0.7: GND -1,-0.8 | smd 0.3 x 0.5: IREF(33,34) -6.35,-2; VTHR(24,16) -8.1,-2 | smd 18 x 0.3: VDDA -1,-0.15; VDDD -1,-1.45
PA = smd 18 x 0.8: P$1 -9,-0.4; P$2 -9,-3.6 | smd 0.15 x 2: P$3 -17.85,-2; P$4 -17.55,-2; P$5 -17.25,-2; P$6 -16.95,-2; P$7 -16.65,-2; P$8 -16.35,-2; P$9 -16.05,-2; P$10 -15.75,-2; P$11 -15.45,-2; P$12 -15.15,-2; P$13 -14.85,-2; P$14 -14.55,-2; P$15 -14.25,-2; P$16 -13.95,-2; P$17 -13.65,-2; P$18 -13.35,-2; P$19 -13.05,-2; P$20 -12.75,-2; P$21 -12.45,-2; P$22 -12.15,-2; P$23 -11.85,-2; P$24 -11.55,-2; P$25 -11.25,-2; P$26 -10.95,-2; P$27 -10.65,-2; P$28 -10.35,-2; P$29 -10.05,-2; P$30 -9.75,-2; P$31 -9.45,-2; P$32 -9.15,-2; P$33 -8.85,-2; P$34 -8.55,-2; P$35 -8.25,-2; P$36 -7.95,-2; P$37 -7.65,-2; P$38 -7.35,-2; P$39 -7.05,-2; P$40 -6.75,-2; P$41 -6.45,-2; P$42 -6.15,-2; P$43 -5.85,-2; P$44 -5.55,-2; P$45 -5.25,-2; P$46 -4.95,-2; P$47 -4.65,-2; P$48 -4.35,-2; P$49 -4.05,-2; P$50 -3.75,-2; P$51 -3.45,-2; P$52 -3.15,-2; P$53 -2.85,-2; P$54 -2.55,-2; P$55 -2.25,-2; P$56 -1.95,-2; P$57 -1.65,-2; P$58 -1.35,-2; P$59 -1.05,-2; P$60 -0.75,-2; P$71 -0.45,-2; P$72 -0.15,-2 | drill 0.3 pad 0.7: P$61 -17,-0.4; P$62 -13,-0.4; P$63 -9,-0.4; P$64 -5,-0.4; P$65 -1,-0.4; P$66 -17,-3.6; P$67 -13,-3.6; P$68 -9,-3.6; P$69 -5,-3.6; P$70 -1,-3.6
5566-8 = drill 1.4 square: 1 6.3,-2.75; 2 2.1,-2.75; 3 -2.1,-2.75; 4 -6.3,-2.75; 5 6.3,2.75; 6 2.1,2.75; 7 -2.1,2.75; 8 -6.3,2.75
RJ45-NO-SHIELD = drill 0.9 pad 1.4: 1 -4.445,6.35; 2 -3.175,8.89; 3 -1.905,6.35; 4 -0.635,8.89; 5 0.635,6.35; 6 1.905,8.89; 7 3.175,6.35; 8 4.445,8.89 | hole 3.251: -5.715,0; 5.715,0

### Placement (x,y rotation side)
BACKPLANE  52.51,74.5 0 top
C1  56.31,84.8 0 top
C2  56.31,80 0 top
C3  20.01,65.1 0 bottom
C4  20.01,62.9 0 bottom
C5  20.01,60 0 bottom
C6  20.01,58.6 0 bottom
C7  20.01,45.1 0 bottom
C8  20.01,42.9 0 bottom
C9  20.01,40 0 bottom
C10  20.01,38.6 0 bottom
C11  85.01,54.9 180 bottom
C12  85.01,57.1 180 bottom
C13  85.01,60.2 180 bottom
C14  85.01,61.5 180 bottom
C15  85.01,34.9 180 bottom
C16  85.01,37.1 180 bottom
C17  85.01,40 180 bottom
C18  85.01,41.4 180 bottom
C19  22.51,86.8 90 bottom
C20  20.91,86.8 90 bottom
C21  22.61,19.8 270 bottom
C22  24.21,19.8 270 bottom
C23  84.11,13.2 270 bottom
C24  82.51,13.2 270 bottom
C25  82.41,80.1 90 bottom
C26  80.91,80.1 90 bottom
C27  17.91,83 90 bottom
C28  19.41,83 90 bottom
C29  19.61,15.9 270 bottom
C30  21.11,15.9 270 bottom
C31  87.01,17 270 bottom
C32  85.51,17 270 bottom
C33  85.41,84.1 90 bottom
C34  83.91,84.1 90 bottom
C35  24.01,72.2 90 bottom
C36  22.51,52.2 90 bottom
C37  22.41,72.2 90 bottom
C38  22.41,55.7 90 bottom
C39  22.51,49.7 270 bottom
C40  24.01,29.9 270 bottom
C41  20.91,47.3 0 bottom
C42  22.31,29.9 270 bottom
C43  81.01,70.2 90 bottom
C44  82.51,50.2 90 bottom
C45  82.61,70.2 90 bottom
C46  84.11,52.8 180 bottom
C47  82.51,47.7 270 bottom
C48  81.01,27.8 270 bottom
C49  82.61,44.3 270 bottom
C50  82.61,27.8 270 bottom
C51  23.91,76.1 270 top
C52  24.81,26.3 180 top
C53  81.11,23.9 90 top
C54  80.41,73.8 0 top
C55  16.11,79.2 270 bottom
C56  14.41,76.4 270 bottom
C57  18.61,11.8 90 bottom
C58  17.11,11.8 90 bottom
C59  86.41,88.2 270 bottom
C60  87.91,88.2 270 bottom
C61  88.91,20.8 90 bottom
C62  90.61,23.6 90 bottom
C63  6.61,49.7 0 top
C64  15.01,73.3 180 top
C65  15.11,27.3 180 top
C66  12.41,49.7 180 top
C67  89.71,72.7 0 top
C68  98.61,50.3 180 top
C69  92.91,50.3 0 top
C70  90.01,26.5 0 top
H1  32.51,80 0 top
H2  32.51,20 0 top
H3  72.51,80 0 top
H4  72.51,20 0 top
HV  52.51,91 0 top
JP1  7.71,72.7 180 top
JP2  7.71,27.3 180 top
JP3  97.31,72.7 0 top
JP4  97.31,27.3 0 top
JP5  21.81,91 90 top
JP6  21.81,10 90 top
JP7  83.21,91 270 top
JP8  83.21,10 90 top
JP9  5.61,82.9 0 top
JP10  5.61,17.1 180 top
JP11  99.41,82.9 0 top
JP12  99.41,17 180 top
R1  47.41,84.3 270 top
R2  48.81,79.6 0 top
R3  20.01,65.2 180 top
R4  20.01,63 180 top
R5  20.01,60.1 180 top
R6  20.01,58.7 180 top
R7  16.61,62.7 180 top
R8  16.61,61.4 180 top
R9  16.61,60.1 180 top
R10  20.01,66.4 0 top
R11  20.01,67.7 0 top
R12  20.01,45.2 180 top
R13  20.01,43 180 top
R14  20.01,40.1 180 top
R15  20.01,38.7 180 top
R16  16.61,42.7 180 top
R17  16.61,41.4 180 top
R18  16.61,40 180 top
R19  20.01,46.4 0 top
R20  20.01,47.7 0 top
R21  85.01,54.8 0 top
R22  85.01,57 0 top
R23  85.01,60.1 0 top
R24  85.01,61.4 0 top
R25  88.41,57.1 0 top
R26  88.41,58.5 0 top
R27  88.41,59.9 0 top
R28  85.01,53.6 180 top
R29  85.01,52.3 180 top
R30  85.01,34.8 0 top
R31  85.01,37 0 top
R32  85.01,39.9 0 top
R33  85.01,41.3 0 top
R34  88.41,37.3 0 top
R35  88.41,38.6 0 top
R36  88.41,39.9 0 top
R37  85.01,33.5 180 top
R38  85.01,32.2 180 top
R39  15.51,52.2 90 bottom
R40  17.01,52.2 90 bottom
R41  52.51,15.3 180 top
R42  52.51,16.8 180 top
R43  89.21,47.8 270 bottom
R44  87.91,47.8 270 bottom
R45  21.81,84.9 180 bottom
R46  23.41,22.5 180 bottom
R47  83.21,15.1 0 bottom
R48  81.71,77.5 0 bottom
R49  21.11,76.1 90 top
R50  22.51,76.1 90 top
R51  22.81,24 270 top
R52  24.21,24 270 top
R53  83.91,23.9 270 top
R54  82.51,23.9 270 top
R55  82.51,76 90 top
R56  81.01,76 90 top
R57  12.51,52.2 90 bottom
R58  14.01,52.2 90 bottom
R59  52.51,12.1 180 top
R60  52.51,13.7 180 top
R61  92.41,47.8 270 bottom
R62  90.91,47.8 270 bottom
R63  18.71,81.1 180 bottom
R64  20.41,22.5 180 bottom
R65  86.31,18.9 0 bottom
R66  84.81,77.5 0 bottom
R67  18.01,79.7 270 top
R68  19.31,76.1 90 top
R69  19.51,24 270 top
R70  20.91,24 270 top
R71  87.01,19.6 90 top
R72  85.61,23.9 270 top
R73  85.51,76 90 top
R74  84.01,76 90 top
R75  21.01,51 270 bottom
R76  84.01,49 270 bottom
R77  22.11,51 270 top
R78  82.91,49 270 top
R79  20.01,54.9 180 top
R80  20.01,34.9 180 top
R81  85.01,65.1 0 top
R82  85.01,45.1 0 top
R83  12.21,76.4 270 bottom
R84  8.01,19 270 bottom
R85  97.01,81 90 bottom
R86  92.81,23.6 90 bottom
R87  4.01,49.7 90 bottom
R88  52.51,10 180 top
R89  101.01,50.3 270 bottom
R90  20.01,69 0 top
R91  85.01,51 180 top
R92  20.01,48.9 0 top
R93  85.01,30.9 180 top
U$1  24.51,60 270 top
U$2  24.51,40 270 top
U$3  80.51,60 90 top
U$4  80.51,40 90 top
U$5  28.01,65.5 180 top
U$6  28.01,58.5 180 top
U$7  28.01,44.5 180 top
U$8  28.01,51.5 180 top
U$9  28.01,37.5 180 top
U$10  28.01,30.5 180 top
U$11  59.01,65.5 180 top
U$12  59.01,58.5 180 top
U$13  59.01,51.5 180 top
U$14  59.01,44.5 180 top
U$15  59.01,37.5 180 top
U$16  59.01,30.5 180 top
X1  7.56,61 270 top
X2  7.51,39 270 top
X3  97.51,61 90 top
X4  97.51,39 90 top
X6  5.51,83 270 top
X7  5.51,17 270 top
X8  99.51,83 90 top
X9  99.51,17 90 top

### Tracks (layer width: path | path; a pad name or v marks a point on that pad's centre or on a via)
AINJ1  (via drill 0.3)
  Top 0.15: U$1.AINJ(46) 12.76,64.45 11.71,65.5 8.51,65.5 v7.71,66.3
  Bottom 0.3: v7.71,66.3 JP1.2
AINJ2  (via drill 0.3)
  Top 0.15: U$2.AINJ(46) 13.36,44.45 12.41,43.5 7.61,43.5 6.61,42.5 6.61,32.9 v7.71,31.8
  Bottom 0.3: v7.71,31.8 JP2.2
AINJ3  (via drill 0.3)
  Top 0.15: U$3.AINJ(46) 92.26,55.55 93.31,56.6 97.51,56.6 98.41,57.5 98.41,67 v97.41,68
  Bottom 0.3: v97.41,68 97.31,68.1 JP3.2
AINJ4  (via drill 0.3)
  Top 0.15: U$4.AINJ(46) 92.16,35.55 93.31,34.4 96.41,34.4 v97.31,33.5
  Bottom 0.3: v97.31,33.5 JP4.2
C1.1
  Bottom 0.3: X6.1 C20.2
C1.2  (via drill 0.3)
  Top 0.3: v18.21,86.2 22.21,86.2 v23.51,87.5
  Bottom 0.3: X6.2 18.19,86.17 v18.21,86.2 | C19.2 23.46,87.45 v23.51,87.5
C1.4
  Bottom 0.3: X6.4 17.9,83.64 C27.2
C1.5
  Bottom 0.3: X6.5 13.01,83.52 13.01,84.3 13.61,84.9 18.91,84.9 19.31,84.5 19.31,83.75 C28.2
C1.7
  Bottom 0.15: 16.09,79.83 C55.1
  Bottom 0.3: X6.7 16.09,79.83
C1.8
  Bottom 0.15: 14.41,78.55 X6.8
  Bottom 0.3: C56.1 14.41,78.55
C2.1
  Bottom 0.3: C21.2 17.06,19.15 14.81,21.4 11.91,21.4 X7.1
C2.2
  Bottom 0.3: X7.2 16.38,18.2 23.91,18.2 24.11,18.4 24.11,19.05 C22.2
C2.4
  Bottom 0.3: C29.2 19.56,15.3 17.71,15.3 15.41,17.6 14.44,17.6 X7.4
C2.5
  Bottom 0.3: X7.5 15.65,16.37 17.61,14.4 20.71,14.4 21.01,14.7 21.01,15.15 C30.2
C2.7
  Bottom 0.3: X7.7 11.81,13.78 11.81,12.3 13.81,10.3 18.31,10.3 18.51,10.5 18.51,11.05 C57.1
C2.8
  Bottom 0.3: C58.1 15.81,11.15 X7.8
C3.1
  Bottom 0.3: C25.2 87.76,80.75 90.01,78.5 93.11,78.5 X8.1
C3.2
  Bottom 0.3: C26.2 80.91,81.4 81.21,81.7 88.75,81.7 X8.2
C3.4
  Bottom 0.3: C33.2 87.16,84.75 89.51,82.4 90.59,82.4 X8.4
C3.5
  Bottom 0.3: C34.2 83.91,85.3 84.21,85.6 87.71,85.6 89.71,83.6 93.13,83.6 X8.5
C3.7
  Bottom 0.3: C59.1 86.41,89.5 86.71,89.8 90.81,89.8 93.11,87.5 93.11,86.22 X8.7
C3.8
  Bottom 0.3: C60.1 89.22,88.85 X8.8
C4.1
  Bottom 0.3: X9.1 C23.2
C4.2  (via drill 0.3)
  Top 0.3: v86.81,13.8 82.51,13.8 v81.21,12.5
  Bottom 0.3: X9.2 86.84,13.82 v86.81,13.8 | v81.21,12.5 82.46,12.5 C24.2
C4.4
  Bottom 0.3: X9.4 87.03,16.37 C31.2
C4.5
  Bottom 0.3: C32.2 85.51,15.7 86.21,15 91.21,15 91.91,15.7 91.91,17.2 92.35,17.63 X9.5
C4.7
  Bottom 0.3: X9.7 88.94,20.18 C61.1
C4.8
  Bottom 0.3: X9.8 C62.1
CAPM1  (via drill 0.3)
  Top 0.15: U$1.CAPM(47) 12.56,64.15 11.71,65 v7.71,65
  Bottom 0.3: v7.71,65 6.71,66 6.71,68.9 5.21,70.4 5.21,72.66 JP1.3
CAPM2  (via drill 0.3)
  Top 0.15: U$2.CAPM(47) 13.76,44.15 12.71,43.1 7.81,43.1 7.01,42.3 7.01,33.8 v7.71,33.1
  Bottom 0.3: v7.71,33.1 7.41,33.1 6.71,32.4 6.71,29.6 5.31,28.2 5.31,27.44 JP2.3
CAPM3  (via drill 0.3)
  Top 0.15: U$3.CAPM(47) 91.96,55.85 93.11,57 97.31,57 98.01,57.7 98.01,66.2 v97.41,66.8
  Bottom 0.3: v97.41,66.8 98.51,67.9 98.51,70.7 99.85,72.04 JP3.3
CAPM4  (via drill 0.3)
  Top 0.15: U$4.CAPM(47) 92.46,35.85 93.51,34.8 v97.31,34.8
  Bottom 0.3: v97.31,34.8 98.31,33.8 98.31,29.2 99.85,27.66 JP4.3
CLK1+  (via drill 0.3)
  Top 0.15: U$1.CLK+(93) 16.76,57.45 16.51,57.2 v15.51,57.2
  Top 0.3: R49.2 21.21,76.75 v21.21,77.7
  Bottom 0.15: R39.2 v15.51,57.2 14.81,57.9 14.81,70.6 21.21,77 v21.21,77.7 21.21,84.85 R45.1
  Bottom 0.3: R45.1 21.16,85.9 C20.1
CLK1-  (via drill 0.3)
  Top 0.15: U$1.CLK-(92) v16.16,57.75
  Top 0.3: R50.2 22.41,76.75 v22.41,77.7
  Bottom 0.15: R40.2 17.01,53.7 16.16,54.55 v16.16,57.75 15.21,58.7 15.21,70.45 22.41,77.65 v22.41,77.7 22.41,84.85 R45.2
  Bottom 0.3: R45.2 22.46,86.1 C19.1
CLK2+  (via drill 0.3)
  Top 0.15: U$2.CLK+(93) 16.66,37.45 16.41,37.2 v15.51,37.2 | v22.71,21.4 22.71,17.2 24.61,15.3 R41.2
  Top 0.3: R51.2 22.71,23.25 v22.71,21.4
  Bottom 0.15: R39.1 15.51,49.9 14.81,49.2 14.81,37.9 v15.51,37.2 16.21,36.5 16.21,29.95 R51.2 22.81,22.55 R46.1
  Bottom 0.3: 22.81,22.5 R46.1 22.71,22.5 v22.71,21.4 22.71,20.55 C21.1
CLK2-  (via drill 0.3)
  Top 0.15: U$2.CLK-(92) 16.16,37.75 v16.11,37.8 | R42.2 51.11,16.8 50.01,15.7 24.91,15.7 24.11,16.5 v24.11,21.4
  Top 0.3: R52.2 24.11,23.25 v24.11,21.4
  Bottom 0.15: v16.11,37.8 15.21,38.7 15.21,49 17.01,50.8 R40.1 | v16.11,37.8 16.21,37.7 | 24.11,22.55 R46.2 24.06,23.15 23.51,23.7 23.01,23.7 16.61,30.1 16.61,37.3 v16.11,37.8
  Bottom 0.3: R46.2 24.11,22.5 v24.11,21.4 24.11,20.55 C22.1
CLK3+  (via drill 0.3)
  Top 0.15: U$3.CLK+(93) 88.16,62.55 88.51,62.9 v89.41,62.9
  Top 0.3: v82.41,78.5 82.41,76.75 R55.2
  Bottom 0.15: R43.1 89.21,50 90.21,51 90.21,62.1 v89.41,62.9 87.81,64.5 87.81,71.2 82.36,76.65 R48.1
  Bottom 0.3: C25.1 v82.41,78.5 82.41,77.55 R48.1
CLK3-  (via drill 0.3)
  Top 0.15: U$3.CLK-(92) 88.76,62.25 v88.81,62.3
  Top 0.3: v81.01,78.5 R56.2
  Bottom 0.15: R44.1 87.91,49.2 89.81,51.1 89.81,61.3 v88.81,62.3 87.41,63.7 87.41,71 82.11,76.3 81.31,76.3 81.06,76.55 R48.2
  Bottom 0.3: C26.1 81.01,79.35 v81.01,78.5 81.01,77.55 R48.2
CLK4+  (via drill 0.3)
  Top 0.15: U$4.CLK+(93) 88.16,42.55 88.51,42.9 v89.41,42.9 | v83.91,22.3 83.91,20.1 79.11,15.3 R41.1
  Top 0.3: R53.2 v83.91,22.3
  Bottom 0.15: v83.91,22.3 90.61,29 90.61,41.7 v89.41,42.9 89.41,46.95 R43.2
  Bottom 0.3: v83.91,22.3 83.91,15.25 R47.1 83.91,15.05 83.91,14.05 C23.1 83.86,13.85
CLK4-  (via drill 0.3)
  Top 0.15: U$4.CLK-(92) 88.76,42.25 v88.81,42.3 | R42.1 54.01,16.8 55.11,15.7 78.91,15.7 82.51,19.3 v82.51,22.3
  Top 0.3: v82.51,22.3 R54.2
  Bottom 0.15: v82.51,22.3 83.31,23.1 84.11,23.1 90.21,29.2 90.21,40.9 v88.81,42.3 88.81,45.6 87.91,46.5 R44.2
  Bottom 0.3: C24.1 82.56,13.85 R47.2 82.51,15.1 v82.51,22.3
CMD1+  (via drill 0.3)
  Top 0.15: U$1.CMD+(95) 17.16,56.85 16.31,56 v14.31,56
  Top 0.3: R67.2 v18.01,77.7
  Bottom 0.15: R57.2 12.51,53.7 12.91,54.1 13.71,54.1 14.31,54.7 v14.31,56 13.51,56.8 13.51,71.6 18.01,76.1 v18.01,77.7 18.01,81.05 R63.1
  Bottom 0.3: R63.1 18.06,82.2 C27.1
CMD1-  (via drill 0.3)
  Top 0.15: U$1.CMD-(94) 16.96,57.15 16.41,56.6 v14.91,56.6
  Top 0.3: R68.2 v19.31,77.7
  Bottom 0.15: R58.2 14.01,53.7 14.91,54.6 v14.91,56.6 13.91,57.6 13.91,71.5 19.31,76.9 v19.31,77.7 19.31,81.05 R63.2
  Bottom 0.3: R63.2 19.36,82.3 C28.1
CMD2+  (via drill 0.3)
  Top 0.15: U$2.CMD+(95) 17.06,36.85 16.21,36 v14.31,36 | v19.61,17.4 23.71,13.3 49.81,13.3 51.01,12.1 R59.2
  Top 0.3: R69.2 19.61,23.25 v19.61,21.4 v19.61,17.4
  Bottom 0.15: R57.1 12.51,50.5 13.61,49.4 13.61,36.7 v14.31,36 15.01,35.3 15.01,28.7 19.76,23.95 R64.1 19.71,22.55
  Bottom 0.3: 19.71,22.55 19.61,22.55 v19.61,21.4 | C29.1 v19.61,17.4
CMD2-  (via drill 0.3)
  Top 0.15: U$2.CMD-(94) 16.86,37.15 16.31,36.6 v14.91,36.6 | v21.11,17.4 C30.1 23.96,13.7 R60.2
  Top 0.3: v21.11,17.4 v21.11,21.4 21.11,23.15 R70.2
  Bottom 0.15: v14.91,36.6 14.01,37.5 R58.1 | v14.91,36.6 15.01,36.5 | R64.2 21.06,23.25 15.41,28.9 15.41,36.1 v14.91,36.6
  Bottom 0.3: R64.2 21.11,22.5 v21.11,21.4 | C30.1 v21.11,17.4
CMD3+  (via drill 0.3)
  Top 0.15: U$3.CMD+(95) 87.76,63.15 88.71,64.1 v90.61,64.1
  Top 0.3: R73.2 85.41,76.75 v85.41,78.5 v85.41,82.6
  Bottom 0.15: R61.1 92.41,49.2 91.31,50.3 91.31,63.4 v90.61,64.1 89.11,65.6 89.11,72.8 85.41,76.5 85.41,77.45 R66.1
  Bottom 0.3: R66.1 85.41,77.55 v85.41,78.5 | C33.1 v85.41,82.6
CMD3-  (via drill 0.3)
  Top 0.15: U$3.CMD-(94) 87.96,62.85 88.61,63.5 v90.01,63.5
  Top 0.3: R74.2 84.11,76.75 v84.11,78.5 84.11,82.5 v84.01,82.6
  Bottom 0.15: R62.1 90.91,62.6 v90.01,63.5 88.76,64.75 88.76,72.55 84.91,76.4 84.41,76.4 84.16,76.65 R66.2
  Bottom 0.3: R66.2 84.11,77.55 v84.11,78.5 | C34.1 84.01,83.35 v84.01,82.6
CMD4+  (via drill 0.3)
  Top 0.15: U$4.CMD+(95) 87.76,43.15 88.71,44.1 v90.61,44.1 | R59.1 53.71,12.1 54.91,13.3 79.11,13.3 86.06,20.25 R71.2 | v87.01,22.3 87.01,21.2
  Top 0.3: v87.01,22.3 R71.2
  Bottom 0.15: v87.01,22.3 87.01,23.9 91.81,28.7 91.81,42.9 v90.61,44.1 90.61,45.3 91.51,46.2 92.11,46.2 92.41,46.5 R61.2
  Bottom 0.3: C31.1 87.01,18.9 | 87.01,18.9 R65.1 | 87.01,18.9 v87.01,22.3
CMD4-  (via drill 0.3)
  Top 0.15: U$4.CMD-(94) 87.96,42.85 88.61,43.5 v90.01,43.5 | v85.61,22.3 85.61,20.3 79.01,13.7 R60.1
  Top 0.3: v85.61,22.3 R72.2
  Bottom 0.15: v85.61,22.3 85.61,23.1 91.41,28.9 91.41,42.1 v90.01,43.5 90.01,45.6 90.91,46.5 R62.2
  Bottom 0.3: C32.1 85.66,17.65 R65.2 85.61,18.9 v85.61,22.3
DOB1+  (via drill 0.3)
  Top 0.15: U$1.DOB+(103) 17.36,56.05 16.71,55.4 v13.71,55.4
  Bottom 0.15: C55.2 16.11,75.2 12.71,71.8 12.71,56.4 v13.71,55.4
DOB1-  (via drill 0.3)
  Top 0.15: U$1.DOB-(104) 17.56,55.75 16.61,54.8 v13.11,54.8
  Bottom 0.15: C56.2 14.26,75.75 | 14.36,75.7 C56.2 | v13.11,54.8 12.31,55.6 12.31,71.9 14.41,74 C56.2
DOB2+  (via drill 0.3)
  Top 0.15: U$2.DOB+(103) 17.36,36.05 16.71,35.4 v13.71,35.4
  Top 0.3: v18.51,13.4 v18.51,21.4
  Bottom 0.15: v13.71,35.4 14.21,34.9 14.21,28.2 18.51,23.9 v18.51,21.4
  Bottom 0.3: C57.2 18.51,12.55 v18.51,13.4
DOB2-  (via drill 0.3)
  Top 0.15: U$2.DOB-(104) 17.56,35.75 16.61,34.8 v13.11,34.8 | v17.31,13.4 17.41,13.5
  Top 0.3: 17.41,13.5 v17.41,21.4
  Bottom 0.15: v13.11,34.8 13.81,34.1 13.81,28 17.41,24.4 v17.41,21.4
  Bottom 0.3: C58.2 17.31,12.65 v17.31,13.4
DOB3+  (via drill 0.3)
  Top 0.15: U$3.DOB+(103) 87.66,63.95 88.41,64.7 v91.21,64.7
  Top 0.3: v86.41,86.7 86.41,78.6 v86.51,78.5
  Bottom 0.15: v86.51,78.5 86.51,77.2 89.96,73.75 89.96,65.95 v91.21,64.7
  Bottom 0.3: C59.2 v86.41,86.7
DOB3-  (via drill 0.3)
  Top 0.15: U$3.DOB-(104) 87.46,64.25 88.51,65.3 v91.81,65.3
  Top 0.3: v87.91,86.7 v87.91,78.5
  Bottom 0.15: v87.91,78.5 87.91,76.4 90.41,73.9 90.41,66.7 v91.81,65.3
  Bottom 0.3: C60.2 v87.91,86.7
DOB4+  (via drill 0.3)
  Top 0.15: U$4.DOB+(103) 87.66,43.95 88.41,44.7 v91.21,44.7
  Bottom 0.15: C61.2 88.91,24.6 92.51,28.2 92.51,43.4 v91.21,44.7
DOB4-  (via drill 0.3)
  Top 0.15: U$4.DOB-(104) 87.46,44.25 88.51,45.3 v91.81,45.3
  Bottom 0.15: C62.2 90.61,25.8 92.91,28.1 92.91,44.2 v91.81,45.3
GND  (via drill 0.3)
  Top 0.3: R10.1 v18.41,66.4 | R19.1 v18.41,46.4 | R37.1 v86.61,33.5 | R53.1 v83.91,25.4 | C53.1 v81.11,22.3 | v21.11,74.6 R49.1 | C51.1 v23.91,77.7 | v26.31,26.2 25.56,26.2 C52.1 | v19.61,25.6 19.61,24.75 R69.1 | v22.91,25.6 22.91,24.75 R51.1 | R28.1 v86.51,53.6 | v82.51,74.5 R55.1 | R73.1 v85.51,74.5 | C54.1 v79.01,73.8 | v81.21,13.9 86.26,18.95 R71.1 | R67.1 18.06,80.4 v23.21,80.4 | R20.1 v18.41,47.7 | R92.1 v18.41,48.9 | R90.1 v18.41,69 | R11.1 v18.41,67.7 | v86.51,52.3 R29.1 R91.1 | R38.1 v86.61,32.2 | R93.1 v86.61,30.9
  Top 0.5: HV.2 57.71,90.36 C1.2 C2.2
  Top 1: C63.- v9.51,49.7 C66.- | C65.- v12.31,27.3 | v12.21,73.3 C64.- | C70.- v92.81,26.5 | C69.- v95.71,50.3 C68.- | C67.- v92.61,72.7
  other vias: 23.71,61 23.71,69 23.71,65 23.71,57 23.71,53 23.71,49 23.71,45 23.71,41 23.71,37 23.71,33 81.31,31 81.31,35 81.31,39 81.31,43 81.31,47 81.31,51 81.31,55 81.31,59 81.31,63 81.31,67
  pour Bottom: 2.61,99.9 2.61,0.1 102.41,0.1 102.41,99.9 55.11,99.9 55.11,84.8 42.01,84.8 42.01,99.9
HIT1  (via drill 0.3)
  Top 0.15: v7.51,53.3 8.11,52.7 15.51,52.7 v17.71,54.9 R79.2 | v19.11,72.9 17.41,74.7 v12.21,74.7
  Bottom 0.15: v17.71,54.9 17.71,57.6 16.01,59.3 16.01,69.8 v19.11,72.9 | R87.2 4.01,51.6 4.51,52.1 6.31,52.1 v7.51,53.3
  Bottom 0.3: v12.21,74.7 R83.2 10.36,75.75 9.41,76.7 9.41,78.7 6.51,81.6 5.64,81.6 JP9.1
HIT2  (via drill 0.3)
  Top 0.15: R80.2 18.11,34.9 17.01,33.8 v13.11,33.8 12.11,34.8 8.81,34.8 7.91,35.7 v7.91,42 | R88.2 30.51,10 27.51,7 10.31,7 v8.91,8.4 | v13.11,23.7 11.31,23.7 8.01,20.4 v8.01,17.3
  Bottom 0.15: v13.11,33.8 v13.11,23.7 | R84.2 7.99,18.37 | R87.1 4.01,47.9 4.61,47.3 6.31,47.3 6.71,46.9 6.71,43.2 v7.91,42
  Bottom 0.3: 7.99,18.37 JP10.1 | R84.2 v8.01,17.3 8.91,16.4 v8.91,8.4
HIT3  (via drill 0.3)
  Top 0.15: R81.2 86.81,65.1 88.71,67 v91.21,67 93.01,65.2 96.41,65.2 97.11,64.5 v97.11,57.9 | v91.21,76.3 93.81,76.3 97.01,79.5 v97.01,82.8
  Bottom 0.15: v91.21,76.3 v91.21,67 | R89.1 101.01,52.1 100.51,52.6 98.11,52.6 97.11,53.6 v97.11,57.9 97.11,58.4
  Bottom 0.3: JP11.1 97.01,81.63 R85.2 v97.01,82.8
HIT4  (via drill 0.3)
  Top 0.15: R82.2 v87.31,45.1 89.41,47.2 96.91,47.2 v97.51,46.6 | R88.1 74.41,10 77.41,7 94.31,7 v96.11,8.8 | v92.81,25.2 87.31,25.2 v86.11,26.4
  Bottom 0.15: v87.31,45.1 87.31,42.3 89.51,40.1 89.51,29.8 v86.11,26.4 | v97.51,46.6 98.91,48 100.31,48 101.01,48.7 R89.2
  Bottom 0.3: v96.11,8.8 96.11,18.2 | 96.11,18.2 96.11,22.3 94.11,24.3 92.86,24.3 R86.2 v92.81,25.2 | JP12.1 96.18,18.27 96.11,18.2
N$1
  Top 0.5: R2.2 50.23,80 52.41,80 52.51,80 | 52.51,80 C2.1 | BACKPLANE.TP 52.51,80
N$2
  Top 0.5: R2.1 47.39,82.88 R1.2 50.39,82.88 52.31,84.8 C1.1
N$3
  Top 0.5: R1.1 47.41,90.36 HV.1
N$4  (via drill 0.3)
  Top 0.15: U$1.RESET1(45) 21.86,64.75 v21.51,65.1 20.76,65.1 R3.1
  Bottom 0.15: C3.1 v21.51,65.1
N$5  (via drill 0.3)
  Top 0.15: U$1.RESET2(56) v21.51,63 R4.1
  Bottom 0.15: v21.51,63 20.76,63 C4.1
N$6  (via drill 0.3)
  Top 0.15: U$1.RESET3(88) 22.16,58.45 22.11,58.5 22.11,58.9 v21.51,59.5 21.21,59.8 20.56,59.8 R5.1
  Bottom 0.15: C5.1 20.76,59.8 21.21,59.8 v21.51,59.5
N$7  (via drill 0.3)
  Top 0.15: U$1.RESET4(89) 21.86,58.15 v21.51,58.5 20.76,58.5 R6.1
  Bottom 0.15: C6.1 20.66,58.5 v21.51,58.5
N$8
  Top 0.15: U$1.GA0(67) 22.11,61.5 21.71,61.9 18.41,61.9 17.81,62.5 17.46,62.5 R7.1
N$9
  Top 0.15: U$1.GA1(68) 21.96,61.15 21.51,61.6 17.46,61.6 R8.1
N$10
  Top 0.15: U$1.GA2(69) 21.81,60.8 21.31,61.3 19.21,61.3 18.01,60.1 R9.1
N$11
  Top 0.15: U$1.IREF(33,34) 20.71,66.35 R10.2
N$12
  Top 0.15: U$1.VTHR(24,16) 21.71,68.1 21.31,67.7 R11.2
N$13
  Top 0.15: U$1.P$1 21.86,55.35 21.41,54.9 R79.1
N$14
  Top 0.15: U$2.GA0(67) 22.01,41.5 21.71,41.8 18.51,41.8 17.81,42.5 17.46,42.5 R16.1
N$15
  Top 0.15: U$2.GA1(68) 21.86,41.15 21.51,41.5 17.36,41.5 R17.1
N$16
  Top 0.15: U$2.GA2(69) 21.71,40.8 21.31,41.2 19.11,41.2 18.11,40.2 17.46,40.2 R18.1
N$17  (via drill 0.3)
  Top 0.15: U$2.RESET1(45) 21.86,44.75 v21.51,45.1 C7.1 R12.1
  Bottom 0.15: C7.1 v21.51,45.1
N$18  (via drill 0.3)
  Top 0.15: U$2.RESET2(56) v21.51,43 R13.1
  Bottom 0.15: C8.1 R13.1 v21.51,43
N$19  (via drill 0.3)
  Top 0.15: U$2.RESET3(88) 22.16,38.45 22.11,38.5 22.11,38.9 v21.51,39.5 21.21,39.8 20.96,39.8 R14.1
  Bottom 0.15: C9.1 20.66,39.8 21.21,39.8 v21.51,39.5
N$20  (via drill 0.3)
  Top 0.15: U$2.RESET4(89) 21.86,38.15 v21.51,38.5 20.86,38.5 R15.1
  Bottom 0.15: C10.1 20.76,38.5 v21.51,38.5
N$21
  Top 0.15: U$2.P$1 22.06,35.35 21.61,34.9 R80.1
N$22
  Top 0.15: U$3.P$1 83.16,64.65 83.61,65.1 R81.1
N$23
  Top 0.15: U$4.P$1 83.26,44.65 83.61,45 84.26,45 R82.1
N$24
  Top 0.15: U$1.TDAC(11) 21.76,68.55 21.41,68.9 20.76,68.9 R90.2
N$25
  Top 0.15: U$2.IREF(33,34) 20.71,46.35 R19.2
N$26
  Top 0.15: U$2.VTHR(24,16) 21.91,48.1 21.61,47.8 20.76,47.8 R20.2
N$27
  Top 0.15: U$3.TDAC(11) 83.26,51.45 83.61,51.1 84.26,51.1 R91.2
N$28
  Top 0.15: U$2.TDAC(11) 21.86,48.55 21.61,48.8 20.76,48.8 R92.2
N$29
  Top 0.15: U$4.TDAC(11) 83.26,31.45 83.61,31.1 84.16,31.1 R93.2
N$50
  Top 0.15: U$3.GA2(69) 83.31,59.2 83.71,58.8 86.41,58.8 87.21,59.6 87.46,59.6 R27.1
N$56
  Top 0.15: U$3.IREF(33,34) 84.31,53.65 R28.2
N$57
  Top 0.15: U$3.GA1(68) 83.16,58.85 83.61,58.4 87.66,58.4 R26.1
N$58
  Top 0.15: U$3.GA0(67) 83.01,58.5 83.51,58 86.51,58 87.21,57.3 87.56,57.3 R25.1
N$59  (via drill 0.3)
  Top 0.15: U$3.RESET1(45) 83.16,55.25 v83.51,54.9 C11.1 R21.1
  Bottom 0.15: C11.1 v83.51,54.9
N$60  (via drill 0.3)
  Top 0.15: U$3.RESET2(56) v83.51,57 R22.1 C12.1
  Bottom 0.15: C12.1 R22.1 v83.51,57
N$61  (via drill 0.3)
  Top 0.15: U$3.RESET3(88) 82.86,61.55 82.91,61.5 82.91,61.1 v83.51,60.5 83.91,60.1 R23.1
  Bottom 0.15: C13.1 83.81,60.2 v83.51,60.5
N$62  (via drill 0.3)
  Top 0.15: U$3.RESET4(89) 83.26,61.85 v83.51,61.6 84.16,61.6 R24.1
  Bottom 0.15: C14.1 84.26,61.6 v83.51,61.6
N$64
  Top 0.15: U$3.VTHR(24,16) 83.31,51.9 83.61,52.2 84.26,52.2 R29.2
N$73
  Top 0.15: R34.1 87.66,37.4 87.11,37.4 86.41,38.1 83.31,38.1 82.91,38.5 U$4.GA0(67)
N$74
  Top 0.15: R35.1 87.56,38.4 83.51,38.4 83.06,38.85 U$4.GA1(68)
N$75
  Top 0.15: R36.1 87.46,39.6 87.21,39.6 86.31,38.7 83.71,38.7 83.21,39.2 U$4.GA2(69)
N$76  (via drill 0.3)
  Top 0.15: U$4.RESET1(45) 83.16,35.25 v83.51,34.9 C15.1 R30.1
  Bottom 0.15: C15.1 v83.51,34.9
N$77  (via drill 0.3)
  Top 0.15: U$4.RESET2(56) v83.51,37 R31.1
  Bottom 0.15: C16.1 R31.1 v83.51,37
N$78  (via drill 0.3)
  Top 0.15: U$4.RESET3(88) 82.86,41.55 82.91,41.5 82.91,41.1 v83.51,40.5 83.81,40.2 84.36,40.2 R32.1
  Bottom 0.15: C17.1 84.16,40.2 83.81,40.2 v83.51,40.5
N$79  (via drill 0.3)
  Top 0.15: U$4.RESET4(89) 83.16,41.85 v83.51,41.5 84.16,41.5 R33.1
  Bottom 0.15: C18.1 83.61,41.4 v83.51,41.5
N$80
  Top 0.15: U$4.IREF(33,34) 84.21,33.65 R37.2
N$81
  Top 0.15: U$4.VTHR(24,16) 83.31,31.9 83.51,32.1 84.26,32.1 R38.2
NTC1+
  Bottom 0.3: X6.3 10.61,84.91 10.11,85.4 10.11,87.9 11.01,88.8 21.81,88.8 23.01,90 23.01,90.93 JP5.1
NTC1-
  Bottom 0.3: X6.6 10.92,81.09 9.21,82.8 9.21,88.2 10.51,89.5 19.61,89.5 20.41,90.3 20.41,90.87 JP5.2
NTC2+
  Bottom 0.3: JP6.1 23.01,9.93 23.01,9.1 21.91,8 12.91,8 9.91,11 9.91,16.95 X7.3
NTC2-
  Bottom 0.3: X7.6 11.11,15.1 10.51,14.5 10.51,11.3 13.11,8.7 19.81,8.7 20.51,9.4 20.51,9.97 JP6.2
NTC3+
  Bottom 0.3: JP7.1 81.94,91.93 83.31,93.3 91.81,93.3 96.11,89 96.11,84.05 X8.3
NTC3-
  Bottom 0.3: X8.6 94.12,84.91 95.31,86.1 95.31,88.7 91.51,92.5 85.31,92.5 84.61,91.8 84.61,91.13 JP7.2
NTC4+
  Bottom 0.3: X9.3 94.41,13.85 94.41,11.8 91.11,8.5 85.51,8.5 84.48,9.53 JP8.1
NTC4-
  Bottom 0.3: X9.6 94.21,18.91 95.11,18.01 95.11,11.5 91.41,7.8 83.41,7.8 82.01,9.2 82.01,9.93 JP8.2
VDDA1  (via drill 0.3)
  Top 0.3: v24.31,70.6 24.36,70.6 U$1.VDDA 24.36,51.4 v23.71,51.4 | R4.2 v18.41,63 | R3.2 v18.41,65.2 17.21,66.4 17.21,69.2 18.11,70.1 21.21,70.1 21.51,69.8 v22.21,69.8
  Top 1: v19.91,51.6 5.21,51.6 5.11,51.7 | C63.+ 5.11,51.7 | 5.11,51.7 5.11,54.4 X1.1
  Bottom 0.3: v23.71,51.4 22.51,51.4 C36.1 21.11,51.55 R75.1 20.96,51.6 v19.91,51.6 | v18.41,65.2 v18.41,63 | v22.21,69.8 23.51,69.8 v24.31,70.6 24.01,70.9 C35.1
VDDA2  (via drill 0.3)
  Top 0.3: v24.41,31.4 v24.36,31.4 U$2.VDDA 24.36,50.5 v23.71,50.5 | R12.2 v18.41,45.2 17.51,46.1 v17.51,49 | R13.2 v18.41,43
  Top 0.5: 23.01,30 v24.41,31.4
  Top 1: X2.1 7.46,30 16.61,30 | 16.61,30 23.01,30 | C65.+ 16.61,30
  Bottom 0.3: v23.71,50.5 22.66,50.5 C39.1 R75.2 18.86,50.35 v17.51,49 | v18.41,43 v18.41,45.2 | v24.36,31.4 24.01,31.05 C40.1
VDDA3  (via drill 0.3)
  Top 0.3: v81.31,49.5 80.71,49.5 80.66,49.55 U$3.VDDA 80.66,68.55 v80.71,68.6 81.91,69.8 | R21.2 v86.51,54.8 87.31,54 v87.31,51 | R22.2 v86.51,57
  Top 1: X3.1 97.76,69.8 88.21,69.8 | 81.91,69.8 88.01,69.8 88.21,69.8 | C67.+ 88.21,69.8
  Bottom 0.3: v81.31,49.5 82.46,49.5 C44.1 83.91,49.55 R76.1 85.96,49.65 v87.31,51 | v86.51,57 v86.51,54.8 | C43.1 81.01,68.9 v80.71,68.6
VDDA4  (via drill 0.3)
  Top 0.3: R30.2 v86.61,34.8 87.81,33.6 87.81,30.7 86.91,29.8 83.91,29.8 83.51,30.2 v82.91,30.2 | R31.2 v86.61,37 | v80.71,29.4 80.66,29.45 U$4.VDDA 80.66,48.45 80.71,48.5 v81.31,48.5
  Top 1: 100.26,48.4 v85.01,48.4 | X4.1 100.26,48.4 | 100.26,48.4 100.26,50.4 C68.+
  Bottom 0.3: v86.61,34.8 v86.61,37 | v82.91,30.2 81.51,30.2 v80.71,29.4 81.01,29.1 C48.1 | v81.31,48.5 82.36,48.5 C47.1 R76.2 84.01,48.4 v85.01,48.4
VDDD1  (via drill 0.3)
  Top 0.15: R5.2 19.36,60.75 19.61,61 21.11,61 21.81,60.3 23.06,60.3
  Top 0.3: 23.06,54.1 23.06,60.3 U$1.VDDD 23.06,70.55 v23.01,70.6 23.01,71.4 | 23.06,54.1 v22.41,54.1 | R7.2 R8.2 R9.2 15.91,60.05 15.91,59 16.31,58.6 19.26,58.6 R6.2 R5.2 | 23.06,54.1 23.06,51.95 22.76,51.65 R77.1 22.16,51.7 | v21.21,71.4 23.01,71.4 | 23.01,71.4 23.86,72.25 23.86,73.9 | C51.2 23.86,75.4 | 23.86,75.4 23.86,73.9 | R68.1 19.31,74.6 20.11,73.8 23.76,73.8 23.86,73.9 | 23.86,75.4 22.56,75.4 R50.1
  Top 1: v21.21,71.4 16.61,71.4 | 16.61,71.4 13.71,71.4 12.21,69.9 7.41,69.9 X1.4 | C64.+ 16.51,71.5 16.61,71.4
  Bottom 0.3: v22.41,54.1 C38.1 | v23.01,70.6 22.51,70.6 22.41,70.7 C37.1
VDDD2  (via drill 0.3)
  Top 0.15: R14.2 19.36,40.75 19.51,40.9 21.11,40.9 21.71,40.3 23.06,40.3 23.06,40
  Top 0.3: 23.06,47.3 U$2.VDDD 23.06,40 23.06,31.4 v23.01,31.4 v17.31,31.4 | 23.06,47.3 23.06,50.15 22.86,50.35 R77.2 | R77.2 22.16,50.3 | v22.41,47.3 23.06,47.3 | R77.2 21.16,50.35 20.91,50.1 19.91,50.1 | R16.2 R17.2 R18.2 15.96,39.05 16.41,38.6 19.26,38.6 R15.2 R14.2 | R52.1 24.16,24.7 C52.2 v21.61,26.3 20.91,25.6 R70.1
  Top 1: 19.91,50.1 16.01,50.1 15.61,49.7 C66.+ 13.91,48.6 13.21,47.9 7.36,47.9 X2.4
  Bottom 0.3: C41.1 v22.41,47.3 | C42.1 22.31,31.2 22.51,31.4 v23.01,31.4 | v21.61,26.3 17.31,30.6 v17.31,31.4
VDDD3  (via drill 0.3)
  Top 0.15: R23.2 85.66,59.45 85.41,59.2 83.81,59.2 83.41,59.6 81.96,59.6
  Top 0.3: 81.96,52.8 U$3.VDDD 81.96,59.6 81.96,68.55 v81.91,68.6 v86.21,68.6 | 81.96,52.8 81.96,49.85 82.11,49.7 82.86,49.7 R78.1 82.96,49.7 85.01,49.7 | v82.61,52.8 81.96,52.8 | R23.2 R24.2 88.41,61.4 89.06,60.75 R27.2 R26.2 R25.2 | R74.1 84.11,75.25 84.11,74.3 v83.61,73.8 C54.2 81.06,75.3 R56.1
  Top 1: X3.4 97.76,52.2 91.91,52.2 91.41,51.7 C69.+ 89.41,50.3 88.81,49.7 85.01,49.7
  Bottom 0.3: C46.1 v82.61,52.8 | C45.1 82.61,68.9 82.31,68.6 v81.91,68.6 | v83.61,73.8 86.21,71.2 v86.21,68.6
VDDD4  (via drill 0.3)
  Top 0.15: R32.2 85.66,39.25 85.51,39.1 83.81,39.1 83.21,39.7 81.96,39.7 U$4.VDDD
  Top 0.3: R32.2 R33.2 88.71,41.3 89.06,40.95 R36.2 R35.2 R34.2 | v83.71,28.5 82.01,28.5 | 82.01,28.5 v82.01,29.4 81.96,29.45 U$4.VDDD | 82.01,28.5 81.11,27.6 81.11,26.4 | R54.1 C53.2 81.11,26.4 | R72.1 85.61,25.6 84.81,26.4 81.11,26.4 | 82.66,48.35 R78.2 82.86,48.3 82.11,48.3 81.96,48.15 81.96,45.8 | 81.96,39.7 81.96,45.8 | v82.61,45.8 81.96,45.8
  Top 1: X4.4 97.66,30.1 93.11,30.1 91.51,28.5 88.71,28.5 88.51,28.5 | 88.51,28.5 v83.71,28.5 | C70.+ 88.51,28.5
  Bottom 0.3: v82.01,29.4 82.41,29.4 82.61,29.2 C50.1 | v82.61,45.8 C49.1

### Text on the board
Top: T1 | T3 | HV | + | + | + | T2 | T4 | Quad Pixel Rigid Board V1.0 | Liverpool University I.T. Nov 2012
